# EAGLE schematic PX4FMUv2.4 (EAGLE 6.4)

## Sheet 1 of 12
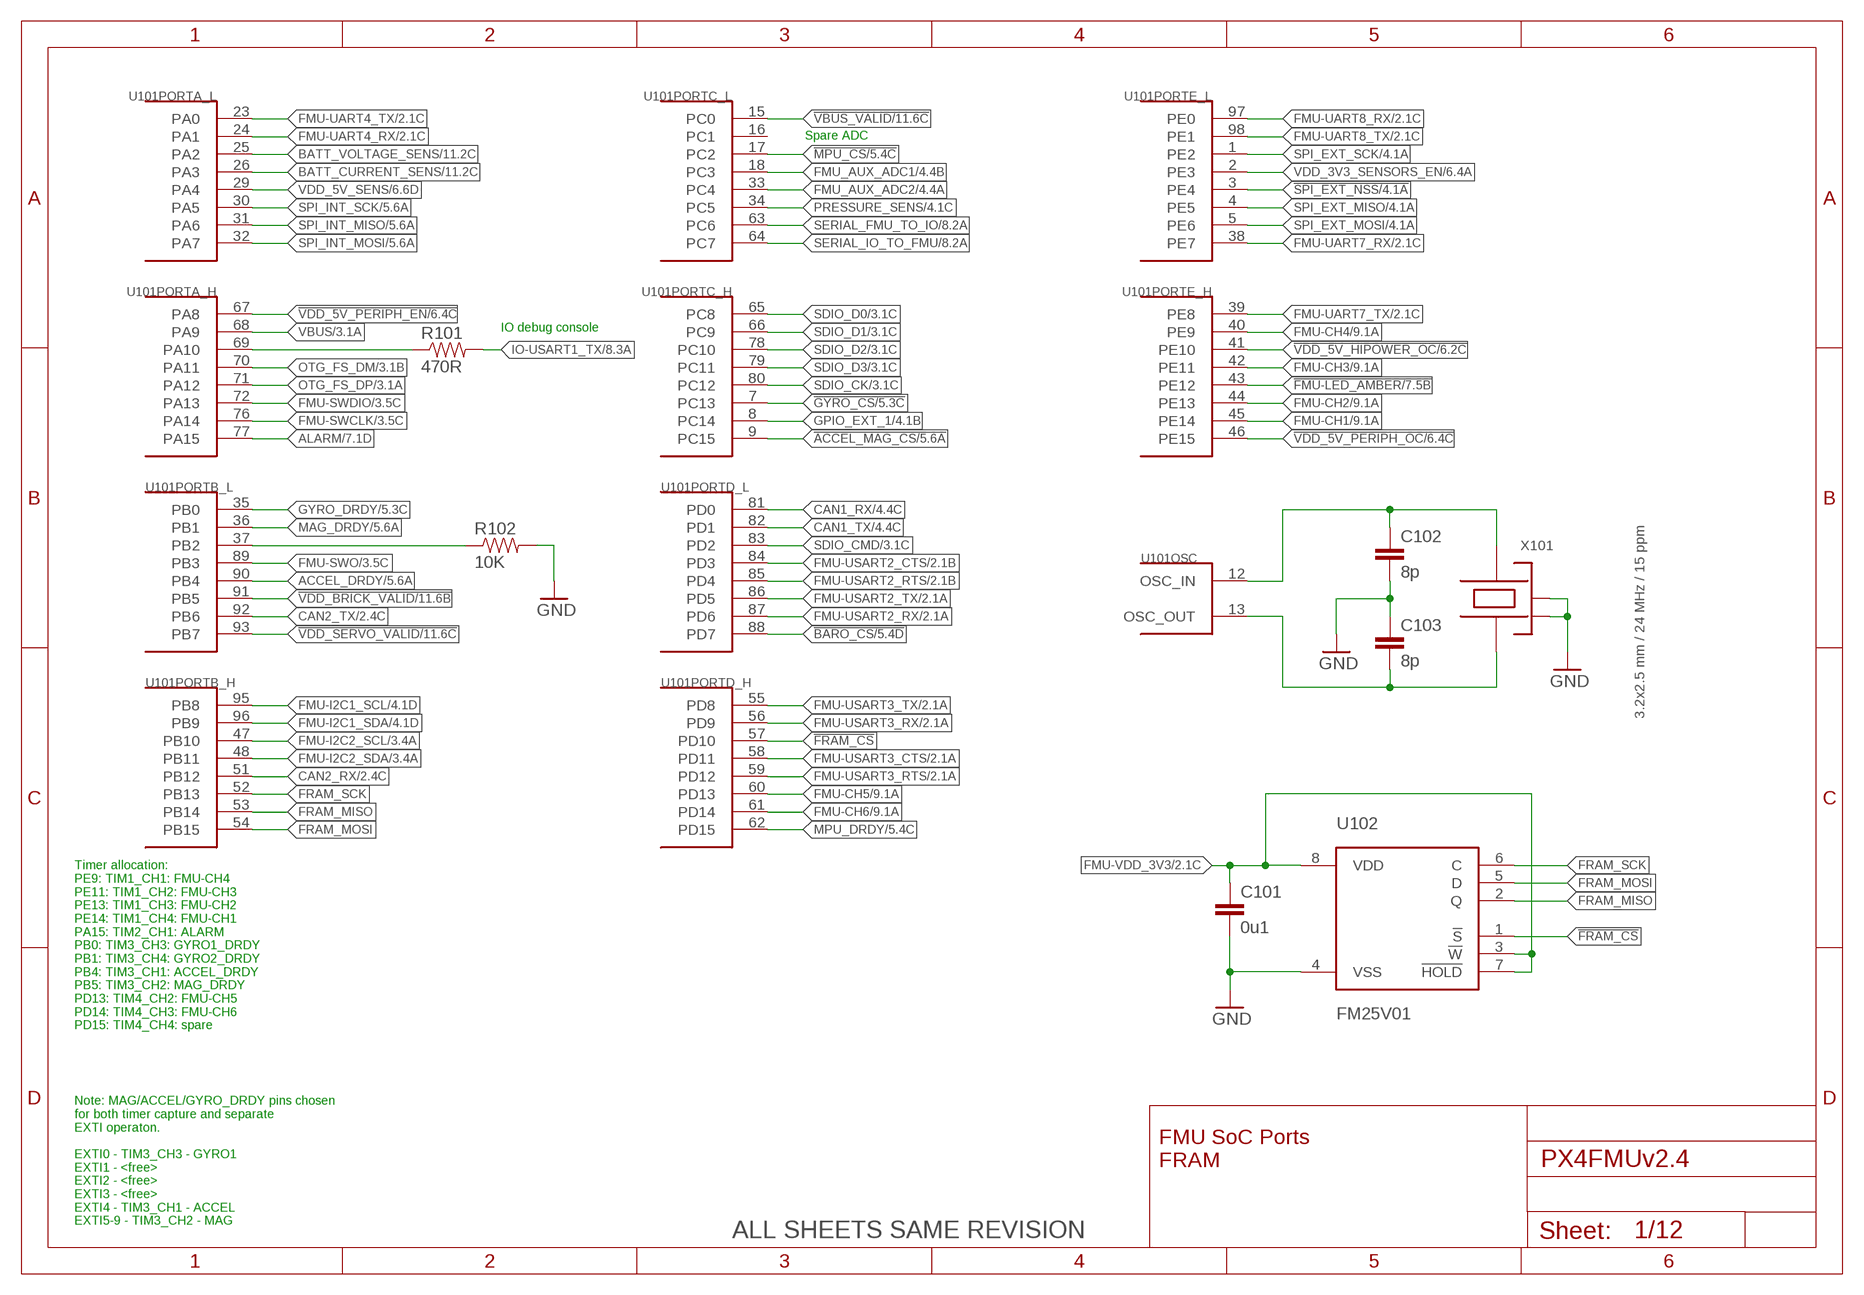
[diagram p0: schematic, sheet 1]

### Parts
C101  0u1  CAP0402  [0402-CAP]
C102  8p  CAP0402  [0402-CAP]
C103  8p  CAP0402  [0402-CAP]
R101  470R  RESISTOR0402-RES  [0402-RES]
R102  10K  RESISTOR0402-RES  [0402-RES]
U101  STM32F4X7VX  [TQFP100]
U102  FM25V01  [SO08]
X101  3.2x2.5 mm / 24 MHz / 15 ppm  OSCILLATOR-3.2X2.5  [OSCILLATOR-3.2X2.5]

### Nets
!ACCEL_MAG_CS: U101.9(PORTC_H:PC15) ; also sheet 5
!BARO_CS: U101.88(PORTD_L:PD7) ; also sheet 5
!FMU-LED_AMBER: U101.43(PORTE_H:PE12) ; also sheet 7
!FRAM_CS: U101.57(PORTD_H:PD10) U102.1(!S)
!GYRO_CS: U101.7(PORTC_H:PC13) ; also sheet 5
!MPU_CS: U101.17(PORTC_L:PC2) ; also sheet 5
!SPI_EXT_NSS: U101.3(PORTE_L:PE4) ; also sheet 4
!VBUS_VALID: U101.15(PORTC_L:PC0) ; also sheet 11,12
!VDD_5V_HIPOWER_OC: U101.41(PORTE_H:PE10) ; also sheet 6
!VDD_5V_PERIPH_EN: U101.67(PORTA_H:PA8) ; also sheet 6
!VDD_5V_PERIPH_OC: U101.46(PORTE_H:PE15) ; also sheet 6
!VDD_BRICK_VALID: U101.91(PORTB_L:PB5) ; also sheet 11,12
!VDD_SERVO_VALID: U101.93(PORTB_L:PB7) ; also sheet 11,12
ACCEL_DRDY: U101.90(PORTB_L:PB4) ; also sheet 5
ALARM: U101.77(PORTA_H:PA15) ; also sheet 7
BATT_CURRENT_SENS: U101.26(PORTA_L:PA3) ; also sheet 11
BATT_VOLTAGE_SENS: U101.25(PORTA_L:PA2) ; also sheet 11
CAN1_RX: U101.81(PORTD_L:PD0) ; also sheet 4
CAN1_TX: U101.82(PORTD_L:PD1) ; also sheet 4
CAN2_RX: U101.51(PORTB_H:PB12) ; also sheet 2
CAN2_TX: U101.92(PORTB_L:PB6) ; also sheet 2
FMU-CH1: U101.45(PORTE_H:PE14) ; also sheet 9
FMU-CH2: U101.44(PORTE_H:PE13) ; also sheet 9
FMU-CH3: U101.42(PORTE_H:PE11) ; also sheet 9
FMU-CH4: U101.40(PORTE_H:PE9) ; also sheet 9
FMU-CH5: U101.60(PORTD_H:PD13) ; also sheet 9
FMU-CH6: U101.61(PORTD_H:PD14) ; also sheet 9
FMU-I2C1_SCL: U101.95(PORTB_H:PB8) ; also sheet 4
FMU-I2C1_SDA: U101.96(PORTB_H:PB9) ; also sheet 4
FMU-I2C2_SCL: U101.47(PORTB_H:PB10) ; also sheet 3,7
FMU-I2C2_SDA: U101.48(PORTB_H:PB11) ; also sheet 3,7
FMU-SWCLK: U101.76(PORTA_H:PA14) ; also sheet 3
FMU-SWDIO: U101.72(PORTA_H:PA13) ; also sheet 3
FMU-SWO: U101.89(PORTB_L:PB3) ; also sheet 3
FMU-UART4_RX: U101.24(PORTA_L:PA1) ; also sheet 2
FMU-UART4_TX: U101.23(PORTA_L:PA0) ; also sheet 2
FMU-UART7_RX: U101.38(PORTE_L:PE7) ; also sheet 2
FMU-UART7_TX: U101.39(PORTE_H:PE8) ; also sheet 2
FMU-UART8_RX: U101.97(PORTE_L:PE0) ; also sheet 2
FMU-UART8_TX: U101.98(PORTE_L:PE1) ; also sheet 2
FMU-USART2_CTS: U101.84(PORTD_L:PD3) ; also sheet 2
FMU-USART2_RTS: U101.85(PORTD_L:PD4) ; also sheet 2
FMU-USART2_RX: U101.87(PORTD_L:PD6) ; also sheet 2
FMU-USART2_TX: U101.86(PORTD_L:PD5) ; also sheet 2
FMU-USART3_CTS: U101.58(PORTD_H:PD11) ; also sheet 2
FMU-USART3_RTS: U101.59(PORTD_H:PD12) ; also sheet 2
FMU-USART3_RX: U101.56(PORTD_H:PD9) ; also sheet 2
FMU-USART3_TX: U101.55(PORTD_H:PD8) ; also sheet 2
FMU-VDD_3V3 [power]: C101.P$1 U102.3(!W) U102.7(!HOLD) U102.8(VDD) ; also sheet 2,3,4,6,7,9,12
FMU_AUX_ADC1: U101.18(PORTC_L:PC3) ; also sheet 4
FMU_AUX_ADC2: U101.33(PORTC_L:PC4) ; also sheet 4
FRAM_MISO: U101.53(PORTB_H:PB14) U102.2(Q)
FRAM_MOSI: U101.54(PORTB_H:PB15) U102.5(D)
FRAM_SCK: U101.52(PORTB_H:PB13) U102.6(C)
GND [power]: C101.P$2 C102.P$2 C103.P$1 R102.P$2 U102.4(VSS) X101.2(NC_2) X101.4(NC_4) ; also sheet 2,3,4,5,6,7,8,9,10,11,12
GPIO_EXT_1: U101.8(PORTC_H:PC14) ; also sheet 4
GYRO_DRDY: U101.35(PORTB_L:PB0) ; also sheet 5
IO-USART1_TX: R101.P$2 ; also sheet 8
MAG_DRDY: U101.36(PORTB_L:PB1) ; also sheet 5
MPU_DRDY [power]: U101.62(PORTD_H:PD15) ; also sheet 5
N$1: C103.P$2 U101.13(OSC:OSC_OUT) X101.1
N$2: C102.P$1 U101.12(OSC:OSC_IN) X101.3
N$23: R101.P$1 U101.69(PORTA_H:PA10)
OTG_FS_DM: U101.70(PORTA_H:PA11) ; also sheet 3
OTG_FS_DP: U101.71(PORTA_H:PA12) ; also sheet 3
PB2-BOOT1: R102.P$1 U101.37(PORTB_L:PB2)
PRESSURE_SENS: U101.34(PORTC_L:PC5) ; also sheet 4
SDIO_CK: U101.80(PORTC_H:PC12) ; also sheet 3
SDIO_CMD: U101.83(PORTD_L:PD2) ; also sheet 3
SDIO_D0: U101.65(PORTC_H:PC8) ; also sheet 3
SDIO_D1: U101.66(PORTC_H:PC9) ; also sheet 3
SDIO_D2: U101.78(PORTC_H:PC10) ; also sheet 3
SDIO_D3: U101.79(PORTC_H:PC11) ; also sheet 3
SERIAL_FMU_TO_IO: U101.63(PORTC_L:PC6) ; also sheet 8
SERIAL_IO_TO_FMU: U101.64(PORTC_L:PC7) ; also sheet 8
SPI_EXT_MISO: U101.4(PORTE_L:PE5) ; also sheet 4
SPI_EXT_MOSI: U101.5(PORTE_L:PE6) ; also sheet 4
SPI_EXT_SCK: U101.1(PORTE_L:PE2) ; also sheet 4
SPI_INT_MISO: U101.31(PORTA_L:PA6) ; also sheet 5
SPI_INT_MOSI: U101.32(PORTA_L:PA7) ; also sheet 5
SPI_INT_SCK: U101.30(PORTA_L:PA5) ; also sheet 5
VBUS [power]: U101.68(PORTA_H:PA9) ; also sheet 3,11,12
VDD_3V3_SENSORS_EN: U101.2(PORTE_L:PE3) ; also sheet 6
VDD_5V_SENS: U101.29(PORTA_L:PA4) ; also sheet 6
Unconnected: U101.16(PORTC_L:PC1)

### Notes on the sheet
- Spare ADC
- IO debug console
- Timer allocation:
  PE9: TIM1_CH1: FMU-CH4
  PE11: TIM1_CH2: FMU-CH3
  PE13: TIM1_CH3: FMU-CH2
  PE14: TIM1_CH4: FMU-CH1
  PA15: TIM2_CH1: ALARM
  PB0: TIM3_CH3: GYRO1_DRDY
  PB1: TIM3_CH4: GYRO2_DRDY
  PB4: TIM3_CH1: ACCEL_DRDY
  PB5: TIM3_CH2: MAG_DRDY
  PD13: TIM4_CH2: FMU-CH5
  PD14: TIM4_CH3: FMU-CH6
  PD15: TIM4_CH4: spare
- FMU SoC Ports
  FRAM
- Note: MAG/ACCEL/GYRO_DRDY pins chosen
  for both timer capture and separate
  EXTI operaton.
  
  EXTI0 - TIM3_CH3 - GYRO1
  EXTI1 - <free>
  EXTI2 - <free>
  EXTI3 - <free>
  EXTI4 - TIM3_CH1 - ACCEL
  EXTI5-9 - TIM3_CH2 - MAG
- ALL SHEETS SAME REVISION

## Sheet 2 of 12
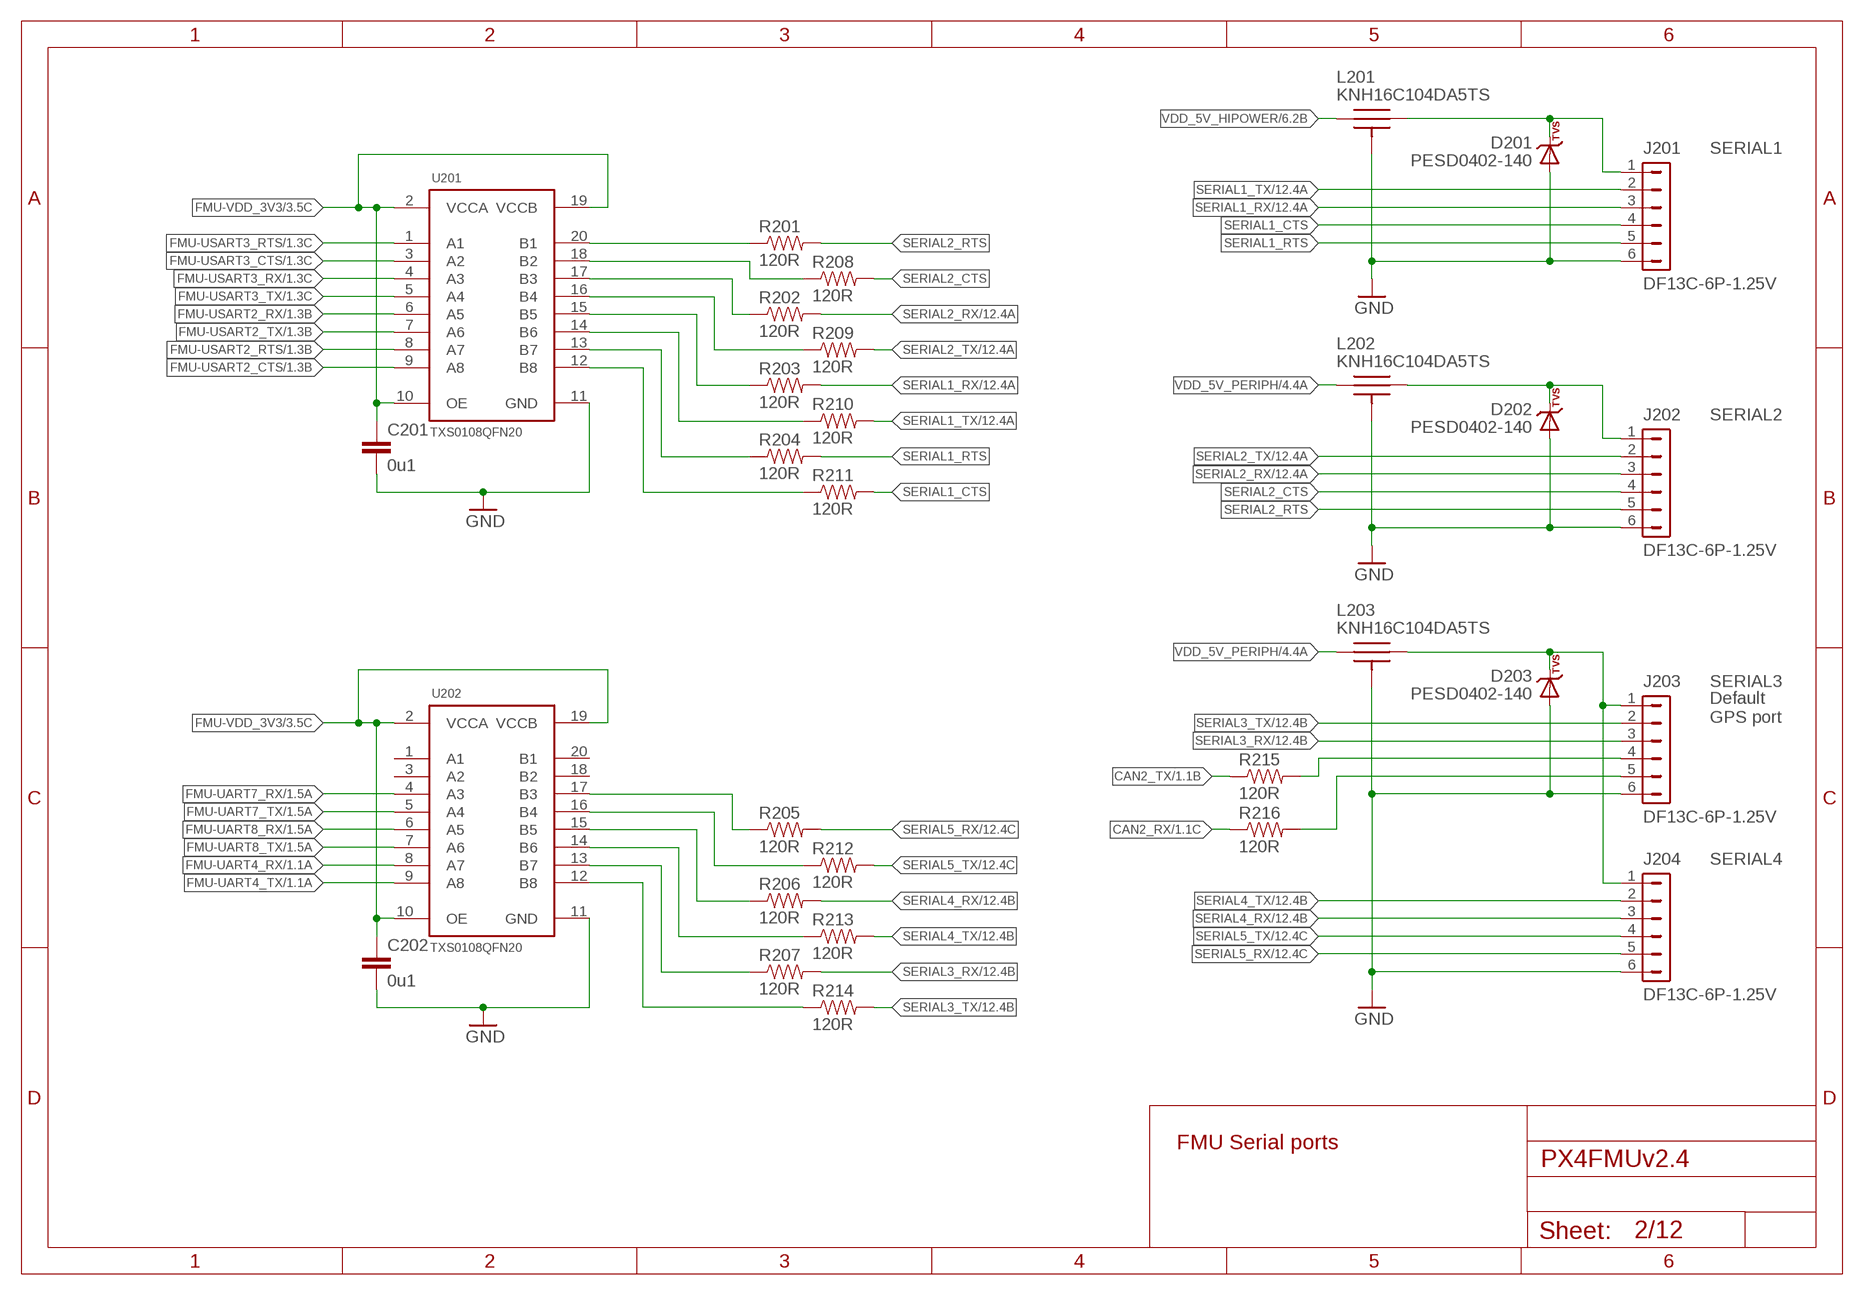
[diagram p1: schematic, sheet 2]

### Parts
C201  0u1  CAP0402  [0402-CAP]
C202  0u1  CAP0402  [0402-CAP]
D201  PESD0402-140  DIODE-TVS  [0402-TVS]
D202  PESD0402-140  DIODE-TVS  [0402-TVS]
D203  PESD0402-140  DIODE-TVS  [0402-TVS]
J201  DF13C-6P-1.25V  DF13-6P-1.25V  [DF13C-6P-1.25V]
J202  DF13C-6P-1.25V  DF13-6P-1.25V  [DF13C-6P-1.25V]
J203  DF13C-6P-1.25V  DF13-6P-1.25V  [DF13C-6P-1.25V]
J204  DF13C-6P-1.25V  DF13-6P-1.25V  [DF13C-6P-1.25V]
L201  KNH16C104DA5TS  [KYOCERA-KNH16-DA]
L202  KNH16C104DA5TS  [KYOCERA-KNH16-DA]
L203  KNH16C104DA5TS  [KYOCERA-KNH16-DA]
R201  120R  RESISTOR0402-RES  [0402-RES]
R202  120R  RESISTOR0402-RES  [0402-RES]
R203  120R  RESISTOR0402-RES  [0402-RES]
R204  120R  RESISTOR0402-RES  [0402-RES]
R205  120R  RESISTOR0402-RES  [0402-RES]
R206  120R  RESISTOR0402-RES  [0402-RES]
R207  120R  RESISTOR0402-RES  [0402-RES]
R208  120R  RESISTOR0402-RES  [0402-RES]
R209  120R  RESISTOR0402-RES  [0402-RES]
R210  120R  RESISTOR0402-RES  [0402-RES]
R211  120R  RESISTOR0402-RES  [0402-RES]
R212  120R  RESISTOR0402-RES  [0402-RES]
R213  120R  RESISTOR0402-RES  [0402-RES]
R214  120R  RESISTOR0402-RES  [0402-RES]
R215  120R  RESISTOR0402-RES  [0402-RES]
R216  120R  RESISTOR0402-RES  [0402-RES]
U201  TXS0108QFN20  [QFN20-RGY]
U202  TXS0108QFN20  [QFN20-RGY]

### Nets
CAN2_RX: R216.P$1 ; also sheet 1
CAN2_TX: R215.P$1 ; also sheet 1
FMU-UART4_RX: U202.8(A7) ; also sheet 1
FMU-UART4_TX: U202.9(A8) ; also sheet 1
FMU-UART7_RX: U202.4(A3) ; also sheet 1
FMU-UART7_TX: U202.5(A4) ; also sheet 1
FMU-UART8_RX: U202.6(A5) ; also sheet 1
FMU-UART8_TX: U202.7(A6) ; also sheet 1
FMU-USART2_CTS: U201.9(A8) ; also sheet 1
FMU-USART2_RTS: U201.8(A7) ; also sheet 1
FMU-USART2_RX: U201.6(A5) ; also sheet 1
FMU-USART2_TX: U201.7(A6) ; also sheet 1
FMU-USART3_CTS: U201.3(A2) ; also sheet 1
FMU-USART3_RTS: U201.1(A1) ; also sheet 1
FMU-USART3_RX: U201.4(A3) ; also sheet 1
FMU-USART3_TX: U201.5(A4) ; also sheet 1
FMU-VDD_3V3 [power]: C201.P$1 C202.P$1 U201.2(VCCA) U201.10(OE) U201.19(VCCB) U202.2(VCCA) U202.10(OE) U202.19(VCCB) ; also sheet 1,3,4,6,7,9,12
GND [power]: C201.P$2 C202.P$2 D201.A D202.A D203.A J201.6 J202.6 J203.6 J204.6 L201.P$3 L201.P$4 L201.P$5 L202.P$3 L202.P$4 L202.P$5 L203.P$3 L203.P$4 L203.P$5 U201.11(GND) U202.11(GND) ; also sheet 1,3,4,5,6,7,8,9,10,11,12
N$5 [power]: D201.C J201.1 L201.P$2
N$14: J203.4 R215.P$2
N$19: J203.5 R216.P$2
N$70: R201.P$1 U201.20(B1)
N$82: R208.P$1 U201.18(B2)
N$83: R202.P$1 U201.17(B3)
N$84: R209.P$1 U201.16(B4)
N$85: R203.P$1 U201.15(B5)
N$86: R210.P$1 U201.14(B6)
N$87: R204.P$1 U201.13(B7)
N$88: R211.P$1 U201.12(B8)
N$89: R207.P$1 U202.13(B7)
N$90: R214.P$1 U202.12(B8)
N$91: R205.P$1 U202.17(B3)
N$92: R212.P$1 U202.16(B4)
N$93: R206.P$1 U202.15(B5)
N$94: R213.P$1 U202.14(B6)
N$100 [power]: D203.C J203.1 J204.1 L203.P$2
N$101 [power]: D202.C J202.1 L202.P$2
SERIAL1_CTS: J201.4 R211.P$2
SERIAL1_RTS: J201.5 R204.P$2
SERIAL1_RX: J201.3 R203.P$2 ; also sheet 12
SERIAL1_TX: J201.2 R210.P$2 ; also sheet 12
SERIAL2_CTS: J202.4 R208.P$2
SERIAL2_RTS: J202.5 R201.P$2
SERIAL2_RX: J202.3 R202.P$2 ; also sheet 12
SERIAL2_TX: J202.2 R209.P$2 ; also sheet 12
SERIAL3_RX: J203.3 R207.P$2 ; also sheet 12
SERIAL3_TX: J203.2 R214.P$2 ; also sheet 12
SERIAL4_RX: J204.3 R206.P$2 ; also sheet 12
SERIAL4_TX: J204.2 R213.P$2 ; also sheet 12
SERIAL5_RX: J204.5 R205.P$2 ; also sheet 12
SERIAL5_TX: J204.4 R212.P$2 ; also sheet 12
VDD_5V_HIPOWER [power]: L201.P$1 ; also sheet 6
VDD_5V_PERIPH [power]: L202.P$1 L203.P$1 ; also sheet 4,6
Unconnected: U202.1(A1) U202.3(A2) U202.18(B2) U202.20(B1)

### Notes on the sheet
- SERIAL1
- SERIAL2
- SERIAL3
- Default 
  GPS port
- SERIAL4
- FMU Serial ports

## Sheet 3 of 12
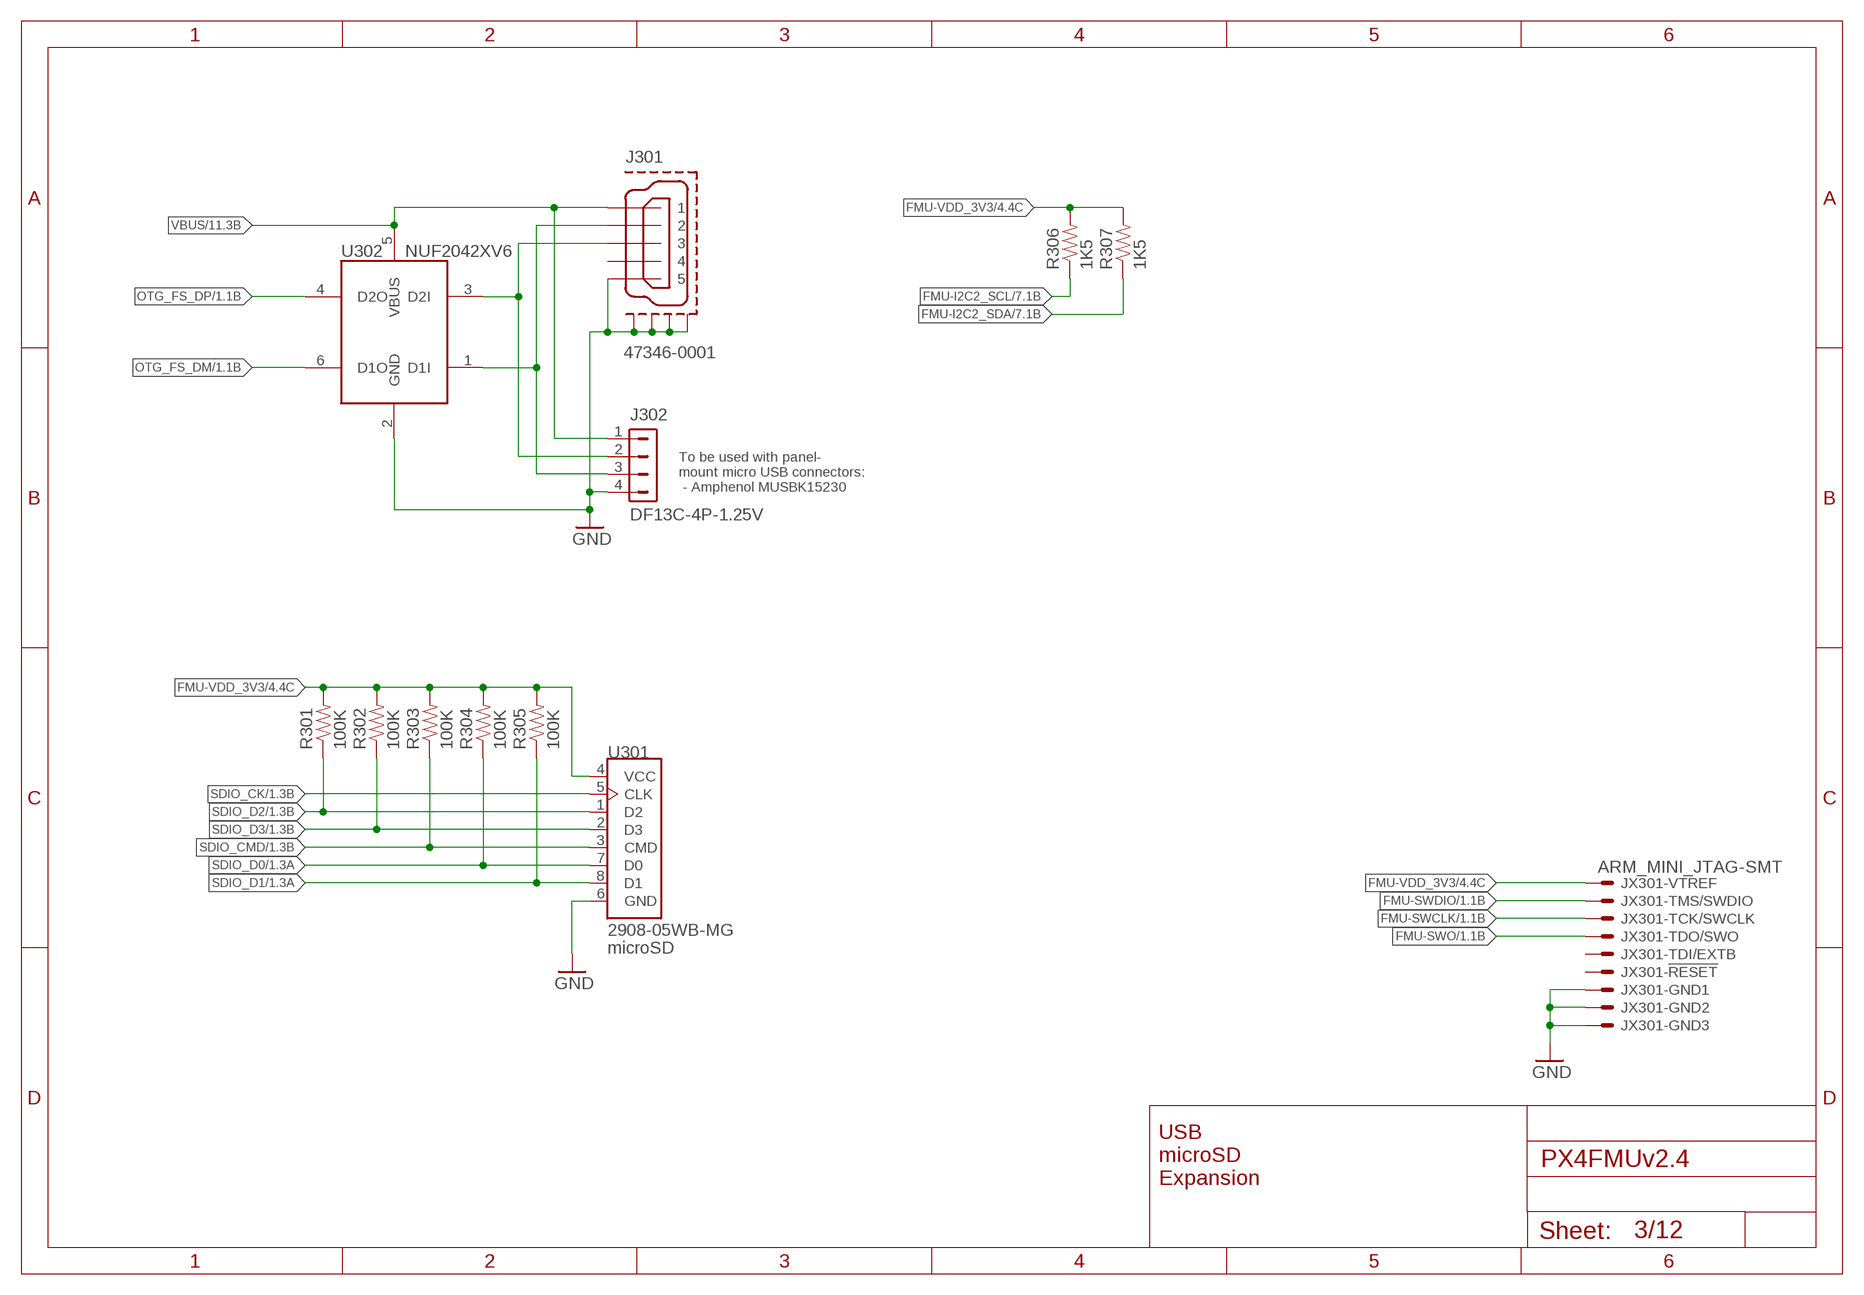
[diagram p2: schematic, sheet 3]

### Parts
J301  47346-0001  MOLEX-47346-0001  [MOLEX-47346-0001]
J302  DF13C-4P-1.25V  DF13-4P-1.25V  [DF13C-4P-1.25V]
JX301  ARM_MINI_JTAG-SMT  [FTSH-105-01-XXX-DV-K]
R301  100K  RESISTOR0402-RES  [0402-RES]
R302  100K  RESISTOR0402-RES  [0402-RES]
R303  100K  RESISTOR0402-RES  [0402-RES]
R304  100K  RESISTOR0402-RES  [0402-RES]
R305  100K  RESISTOR0402-RES  [0402-RES]
R306  1K5  RESISTOR0402-RES  [0402-RES]
R307  1K5  RESISTOR0402-RES  [0402-RES]
U301  2908-05WB-MG  MICROSDSDI  [MICROSD]
U302  NUF2042XV6  [SOT563-6]

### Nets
FMU-I2C2_SCL: R306.P$1 ; also sheet 1,7
FMU-I2C2_SDA: R307.P$1 ; also sheet 1,7
FMU-SWCLK: JX301.4 ; also sheet 1
FMU-SWDIO: JX301.2 ; also sheet 1
FMU-SWO: JX301.6 ; also sheet 1
FMU-VDD_3V3 [power]: JX301.1 R301.P$2 R302.P$2 R303.P$2 R304.P$2 R305.P$2 R306.P$2 R307.P$2 U301.4(VCC) ; also sheet 1,2,4,6,7,9,12
GND [power]: J301.GND J301.GND1 J301.GND2 J301.GND3 J301.GND4 J302.4 JX301.3 JX301.5 JX301.9 U301.6(GND) U302.2(GND) ; also sheet 1,2,4,5,6,7,8,9,10,11,12
OTG_DM1: J301.D- J302.3 U302.1(D1I)
OTG_DP1: J301.D+ J302.2 U302.3(D2I)
OTG_FS_DM: U302.6(D1O) ; also sheet 1
OTG_FS_DP: U302.4(D2O) ; also sheet 1
SDIO_CK: U301.5(CLK) ; also sheet 1
SDIO_CMD: R303.P$1 U301.3(CMD) ; also sheet 1
SDIO_D0: R304.P$1 U301.7(D0) ; also sheet 1
SDIO_D1: R305.P$1 U301.8(D1) ; also sheet 1
SDIO_D2: R301.P$1 U301.1(D2) ; also sheet 1
SDIO_D3: R302.P$1 U301.2(D3) ; also sheet 1
VBUS [power]: J301.VBUS J302.1 U302.5(VBUS) ; also sheet 1,11,12
Unconnected: J301.ID JX301.8 JX301.10

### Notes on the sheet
- To be used with panel-
  mount micro USB connectors:
   - Amphenol MUSBK15230
- microSD
- USB
  microSD
  Expansion

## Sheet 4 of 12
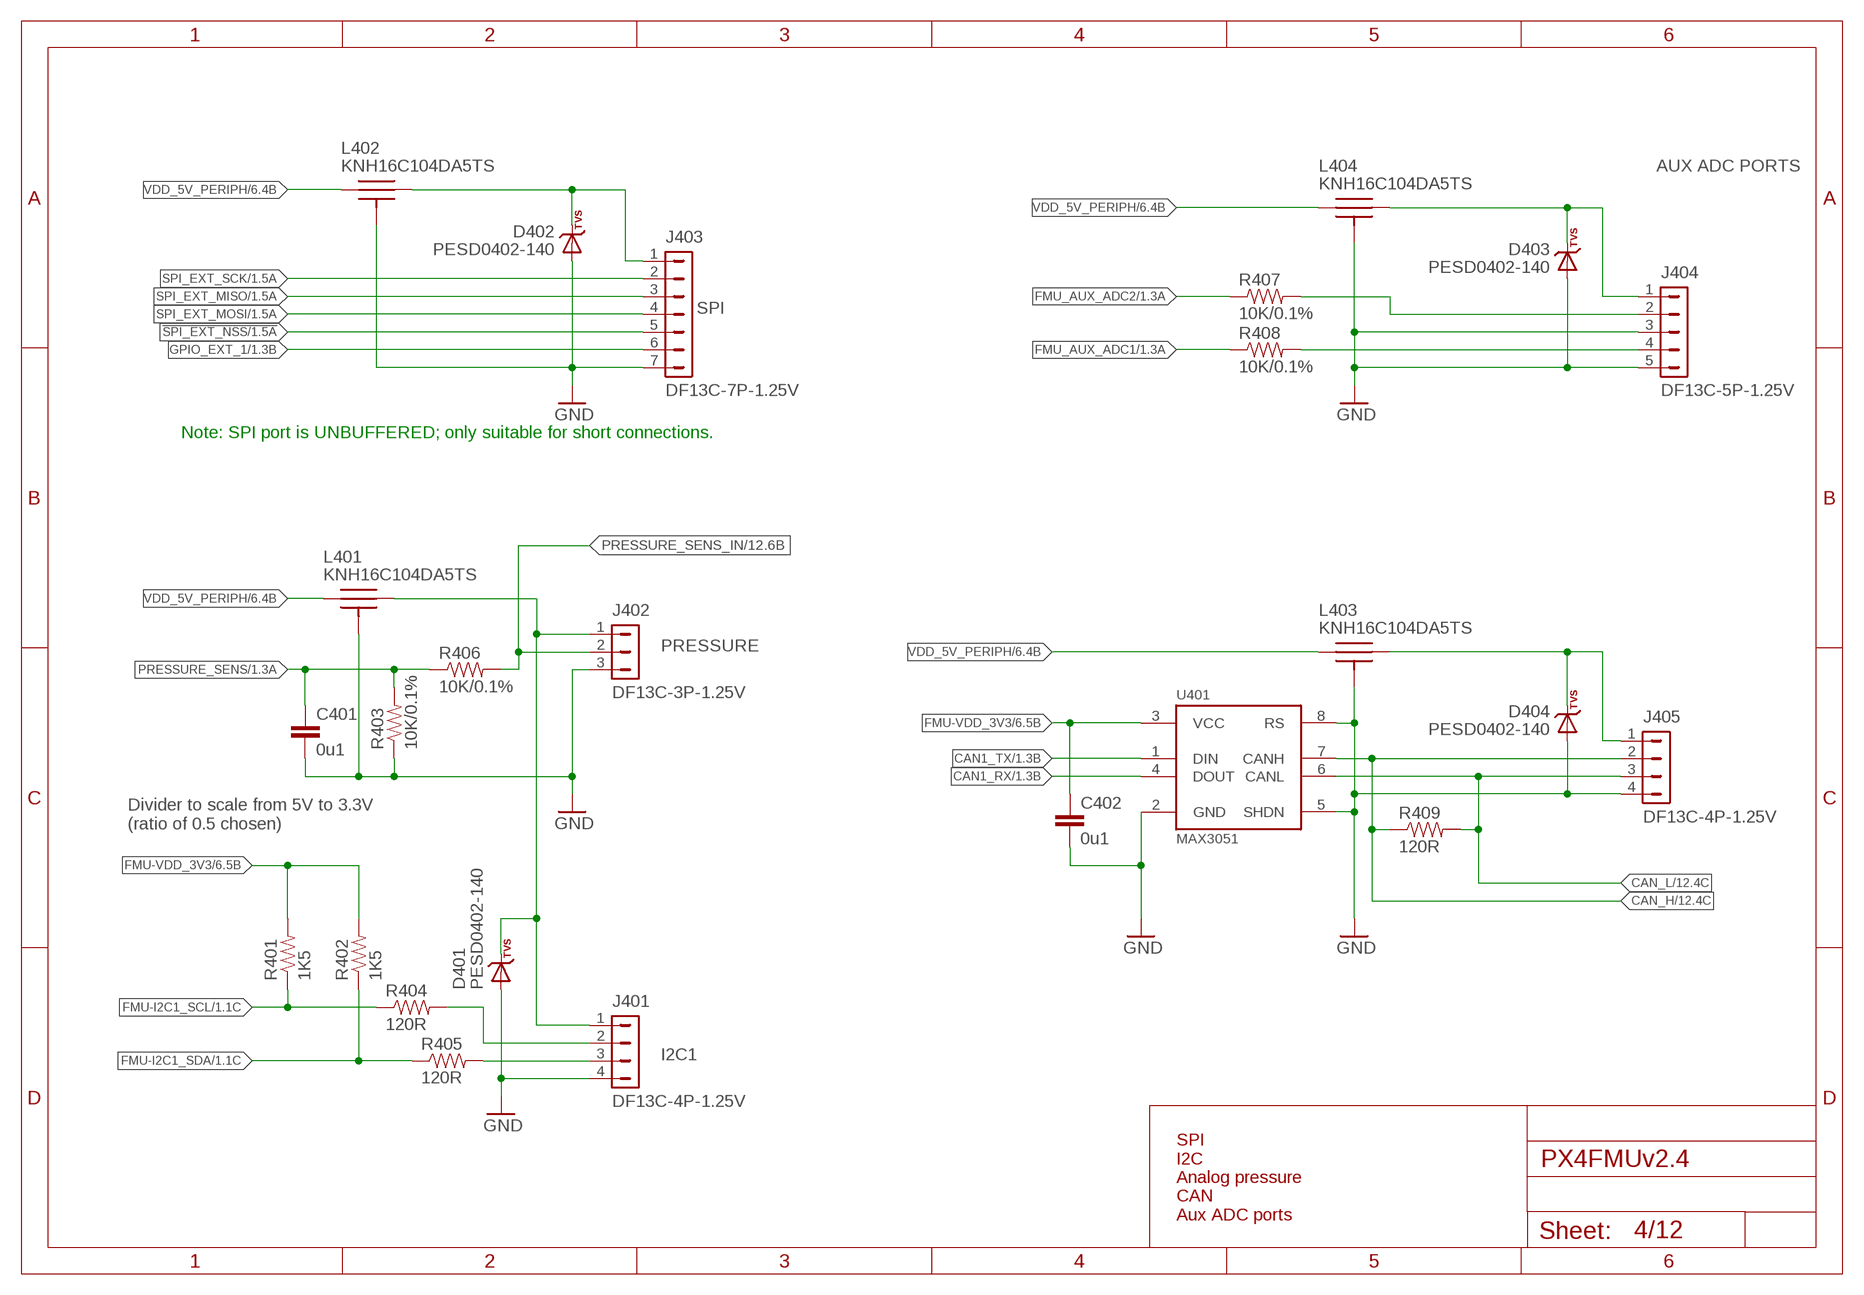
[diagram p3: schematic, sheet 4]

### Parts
C401  0u1  CAP0402  [0402-CAP]
C402  0u1  CAP0402  [0402-CAP]
D401  PESD0402-140  DIODE-TVS  [0402-TVS]
D402  PESD0402-140  DIODE-TVS  [0402-TVS]
D403  PESD0402-140  DIODE-TVS  [0402-TVS]
D404  PESD0402-140  DIODE-TVS  [0402-TVS]
J401  DF13C-4P-1.25V  DF13-4P-1.25V  [DF13C-4P-1.25V]
J402  DF13C-3P-1.25V  DF13-3P-1.25V  [DF13C-3P-1.25V]
J403  DF13C-7P-1.25V  DF13-7P-1.25V  [DF13C-7P-1.25V]
J404  DF13C-5P-1.25V  DF13-5P-1.25V  [DF13C-5P-1.25V]
J405  DF13C-4P-1.25V  DF13-4P-1.25V  [DF13C-4P-1.25V]
L401  KNH16C104DA5TS  [KYOCERA-KNH16-DA]
L402  KNH16C104DA5TS  [KYOCERA-KNH16-DA]
L403  KNH16C104DA5TS  [KYOCERA-KNH16-DA]
L404  KNH16C104DA5TS  [KYOCERA-KNH16-DA]
R401  1K5  RESISTOR0402-RES  [0402-RES]
R402  1K5  RESISTOR0402-RES  [0402-RES]
R403  10K/0.1%  RESISTOR0402-RES  [0402-RES]
R404  120R  RESISTOR0402-RES  [0402-RES]
R405  120R  RESISTOR0402-RES  [0402-RES]
R406  10K/0.1%  RESISTOR0402-RES  [0402-RES]
R407  10K/0.1%  RESISTOR0402-RES  [0402-RES]
R408  10K/0.1%  RESISTOR0402-RES  [0402-RES]
R409  120R  RESISTOR0402-RES  [0402-RES]
U401  MAX3051  MAX3051MAX3051EKA  [SOT23-8]

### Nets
!SPI_EXT_NSS: J403.5 ; also sheet 1
CAN1_RX: U401.4(DOUT) ; also sheet 1
CAN1_TX: U401.1(DIN) ; also sheet 1
CAN_H: J405.2 R409.P$1 U401.7(CANH) ; also sheet 12
CAN_L: J405.3 R409.P$2 U401.6(CANL) ; also sheet 12
FMU-I2C1_SCL: R401.P$1 R404.P$1 ; also sheet 1
FMU-I2C1_SDA: R402.P$1 R405.P$1 ; also sheet 1
FMU-VDD_3V3 [power]: C402.P$1 R401.P$2 R402.P$2 U401.3(VCC) ; also sheet 1,2,3,6,7,9,12
FMU_AUX_ADC1: R408.P$1 ; also sheet 1
FMU_AUX_ADC1_PROT: J404.4 R408.P$2
FMU_AUX_ADC2: R407.P$1 ; also sheet 1
FMU_AUX_ADC2_PROT: J404.2 R407.P$2
GND [power]: C401.P$2 C402.P$2 D401.A D402.A D403.A D404.A J401.4 J402.3 J403.7 J404.3 J404.5 J405.4 L401.P$3 L401.P$4 L401.P$5 L402.P$3 L402.P$4 L402.P$5 L403.P$3 L403.P$4 L403.P$5 L404.P$3 L404.P$4 L404.P$5 R403.P$1 U401.2(GND) U401.5(SHDN) U401.8(RS) ; also sheet 1,2,3,5,6,7,8,9,10,11,12
GPIO_EXT_1: J403.6 ; also sheet 1
N$33: J401.2 R404.P$2
N$37: J401.3 R405.P$2
N$41 [power]: D402.C J403.1 L402.P$2
N$42 [power]: D401.C J401.1 J402.1 L401.P$2
N$48 [power]: D404.C J405.1 L403.P$2
N$98 [power]: D403.C J404.1 L404.P$2
PRESSURE_SENS: C401.P$1 R403.P$2 R406.P$1 ; also sheet 1
PRESSURE_SENS_IN: J402.2 R406.P$2 ; also sheet 12
SPI_EXT_MISO: J403.3 ; also sheet 1
SPI_EXT_MOSI: J403.4 ; also sheet 1
SPI_EXT_SCK: J403.2 ; also sheet 1
VDD_5V_PERIPH [power]: L401.P$1 L402.P$1 L403.P$1 L404.P$1 ; also sheet 2,6

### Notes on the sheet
- AUX ADC PORTS
- SPI
- Note: SPI port is UNBUFFERED; only suitable for short connections.
- PRESSURE
- Divider to scale from 5V to 3.3V
  (ratio of 0.5 chosen)
- I2C1
- SPI
  I2C
  Analog pressure
  CAN
  Aux ADC ports

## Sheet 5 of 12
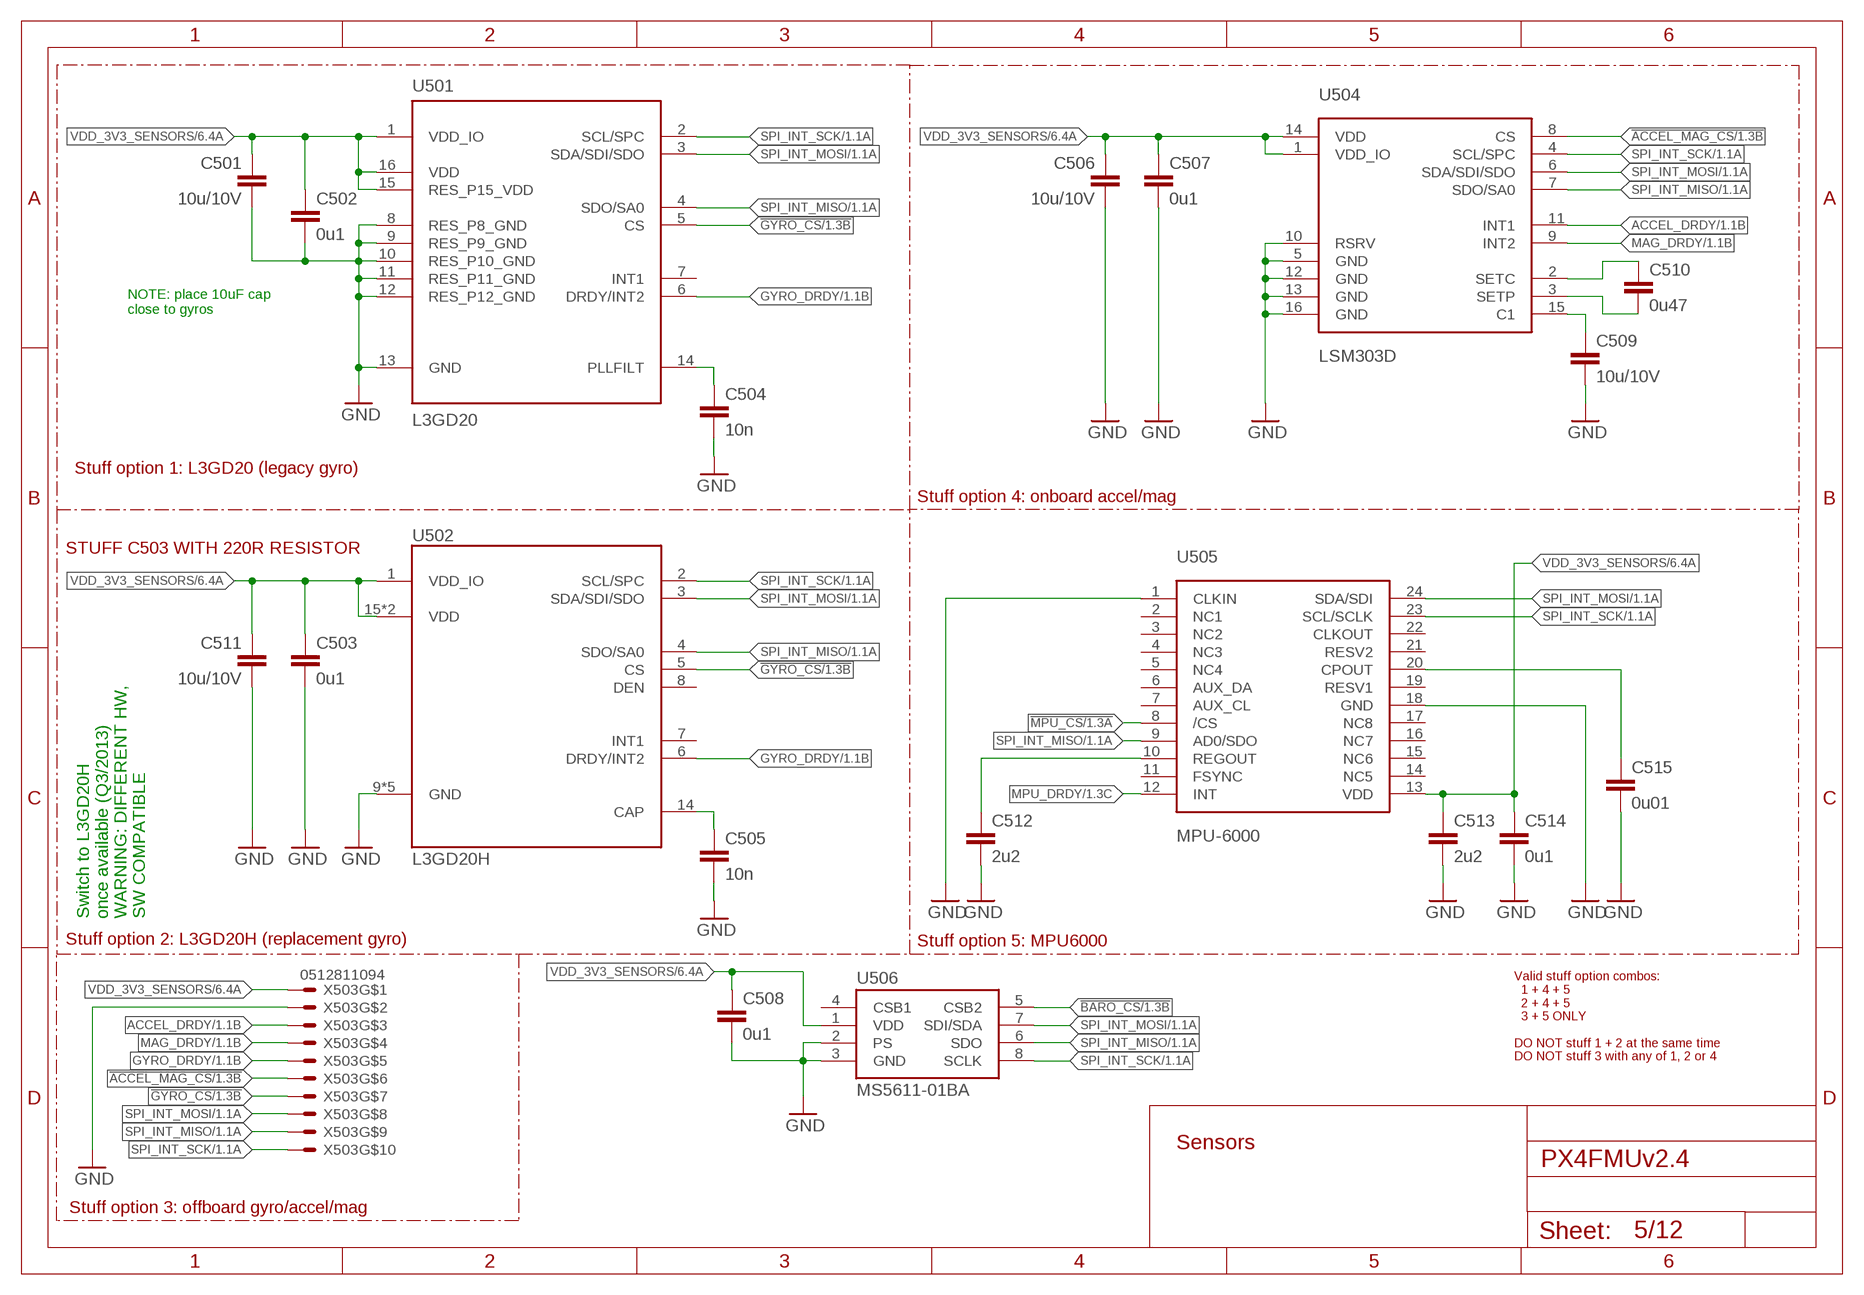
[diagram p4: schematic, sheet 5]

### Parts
C501  10u/10V  CAP0805  [0805-CAP]
C502  0u1  CAP0402  [0402-CAP]
C503  0u1  CAP0402  [0402-CAP]
C504  10n  CAP0402  [0402-CAP]
C505  10n  CAP0402  [0402-CAP]
C506  10u/10V  CAP0805  [0805-CAP]
C507  0u1  CAP0402  [0402-CAP]
C508  0u1  CAP0402  [0402-CAP]
C509  10u/10V  CAP0805  [0805-CAP]
C510  0u47  CAP0402  [0402-CAP]
C511  10u/10V  CAP0805  [0805-CAP]
C512  2u2  CAP0603  [0603-CAP]
C513  2u2  CAP0603  [0603-CAP]
C514  0u1  CAP0402  [0402-CAP]
C515  0u01  CAP0603  [0603-CAP]
U501  L3GD20  L3G4200DH-LL  [L3G4200DH-MAN]
U502  L3GD20H  [LGA-16L]
U504  LSM303D  [LGA-16L]
U505  MPU-6000  [QFN-24]
U506  MS5611-01BA  [MS5611-01BA]
X503  0512811094  CONN_FPC_10RA  [51281-1094]

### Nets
!ACCEL_MAG_CS: U504.8(CS) X503.6 ; also sheet 1
!BARO_CS: U506.5(CSB2) ; also sheet 1
!GYRO_CS: U501.5(CS) U502.5(CS) X503.7 ; also sheet 1
!MPU_CS: U505.8(/CS) ; also sheet 1
ACCEL_DRDY: U504.11(INT1) X503.3 ; also sheet 1
GND [power]: C501.P$2 C502.P$2 C503.P$2 C504.P$2 C505.P$2 C506.P$2 C507.P$2 C508.P$2 C509.P$2 C511.P$2 C512.P$2 C513.P$2 C514.P$2 C515.P$2 U501.8(RES_P8_GND) U501.9(RES_P9_GND) U501.10(RES_P10_GND) U501.11(RES_P11_GND) U501.12(RES_P12_GND) U501.13(GND) U502.9(GND) U502.10(GND) U502.11(GND) U502.12(GND) U502.13(GND) U504.5(GND) U504.10(RSRV) U504.12(GND) U504.13(GND) U504.16(GND) U505.1(CLKIN) U505.18(GND) U506.2(PS) U506.3(GND) X503.2 ; also sheet 1,2,3,4,6,7,8,9,10,11,12
GYRO_DRDY: U501.6(DRDY/INT2) U502.6(DRDY/INT2) X503.5 ; also sheet 1
MAG_DRDY: U504.9(INT2) X503.4 ; also sheet 1
MPU_DRDY [power]: U505.12(INT) ; also sheet 1
N$6: C509.P$1 U504.15(C1)
N$10: C510.P$1 U504.2(SETC)
N$17: C510.P$2 U504.3(SETP)
N$30: C505.P$1 U502.14(CAP)
N$35: C504.P$1 U501.14(PLLFILT)
N$50: C512.P$1 U505.10(REGOUT)
N$51: C515.P$1 U505.20(CPOUT)
SPI_INT_MISO: U501.4(SDO/SA0) U502.4(SDO/SA0) U504.7(SDO/SA0) U505.9(AD0/SDO) U506.6(SDO) X503.9 ; also sheet 1
SPI_INT_MOSI: U501.3(SDA/SDI/SDO) U502.3(SDA/SDI/SDO) U504.6(SDA/SDI/SDO) U505.24(SDA/SDI) U506.7(SDI/SDA) X503.8 ; also sheet 1
SPI_INT_SCK: U501.2(SCL/SPC) U502.2(SCL/SPC) U504.4(SCL/SPC) U505.23(SCL/SCLK) U506.8(SCLK) X503.10 ; also sheet 1
VDD_3V3_SENSORS [power]: C501.P$1 C502.P$1 C503.P$1 C506.P$1 C507.P$1 C508.P$1 C511.P$1 C513.P$1 C514.P$1 U501.1(VDD_IO) U501.15(RES_P15_VDD) U501.16(VDD) U502.1(VDD_IO) U502.15(VDD) U502.16(VDD) U504.1(VDD_IO) U504.14(VDD) U505.13(VDD) U506.1(VDD) X503.1 ; also sheet 6,12
Unconnected: U501.7(INT1) U502.7(INT1) U502.8(DEN) U505.2(NC1) U505.3(NC2) U505.4(NC3) U505.5(NC4) U505.6(AUX_DA) U505.7(AUX_CL) U505.11(FSYNC) U505.14(NC5) U505.15(NC6) U505.16(NC7) U505.17(NC8) U505.19(RESV1) U505.21(RESV2) U505.22(CLKOUT) U506.4(CSB1)

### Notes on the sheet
- NOTE: place 10uF cap
  close to gyros
- Stuff option 1: L3GD20 (legacy gyro)
- Stuff option 4: onboard accel/mag
- STUFF C503 WITH 220R RESISTOR
- Switch to L3GD20H
  once available (Q3/2013)
  WARNING: DIFFERENT HW,
  SW COMPATIBLE
- Stuff option 2: L3GD20H (replacement gyro) | Stuff option 5: MPU6000
- Valid stuff option combos:
    1 + 4 + 5
    2 + 4 + 5
    3 + 5 ONLY
  
  DO NOT stuff 1 + 2 at the same time
  DO NOT stuff 3 with any of 1, 2 or 4
- Sensors
- Stuff option 3: offboard gyro/accel/mag

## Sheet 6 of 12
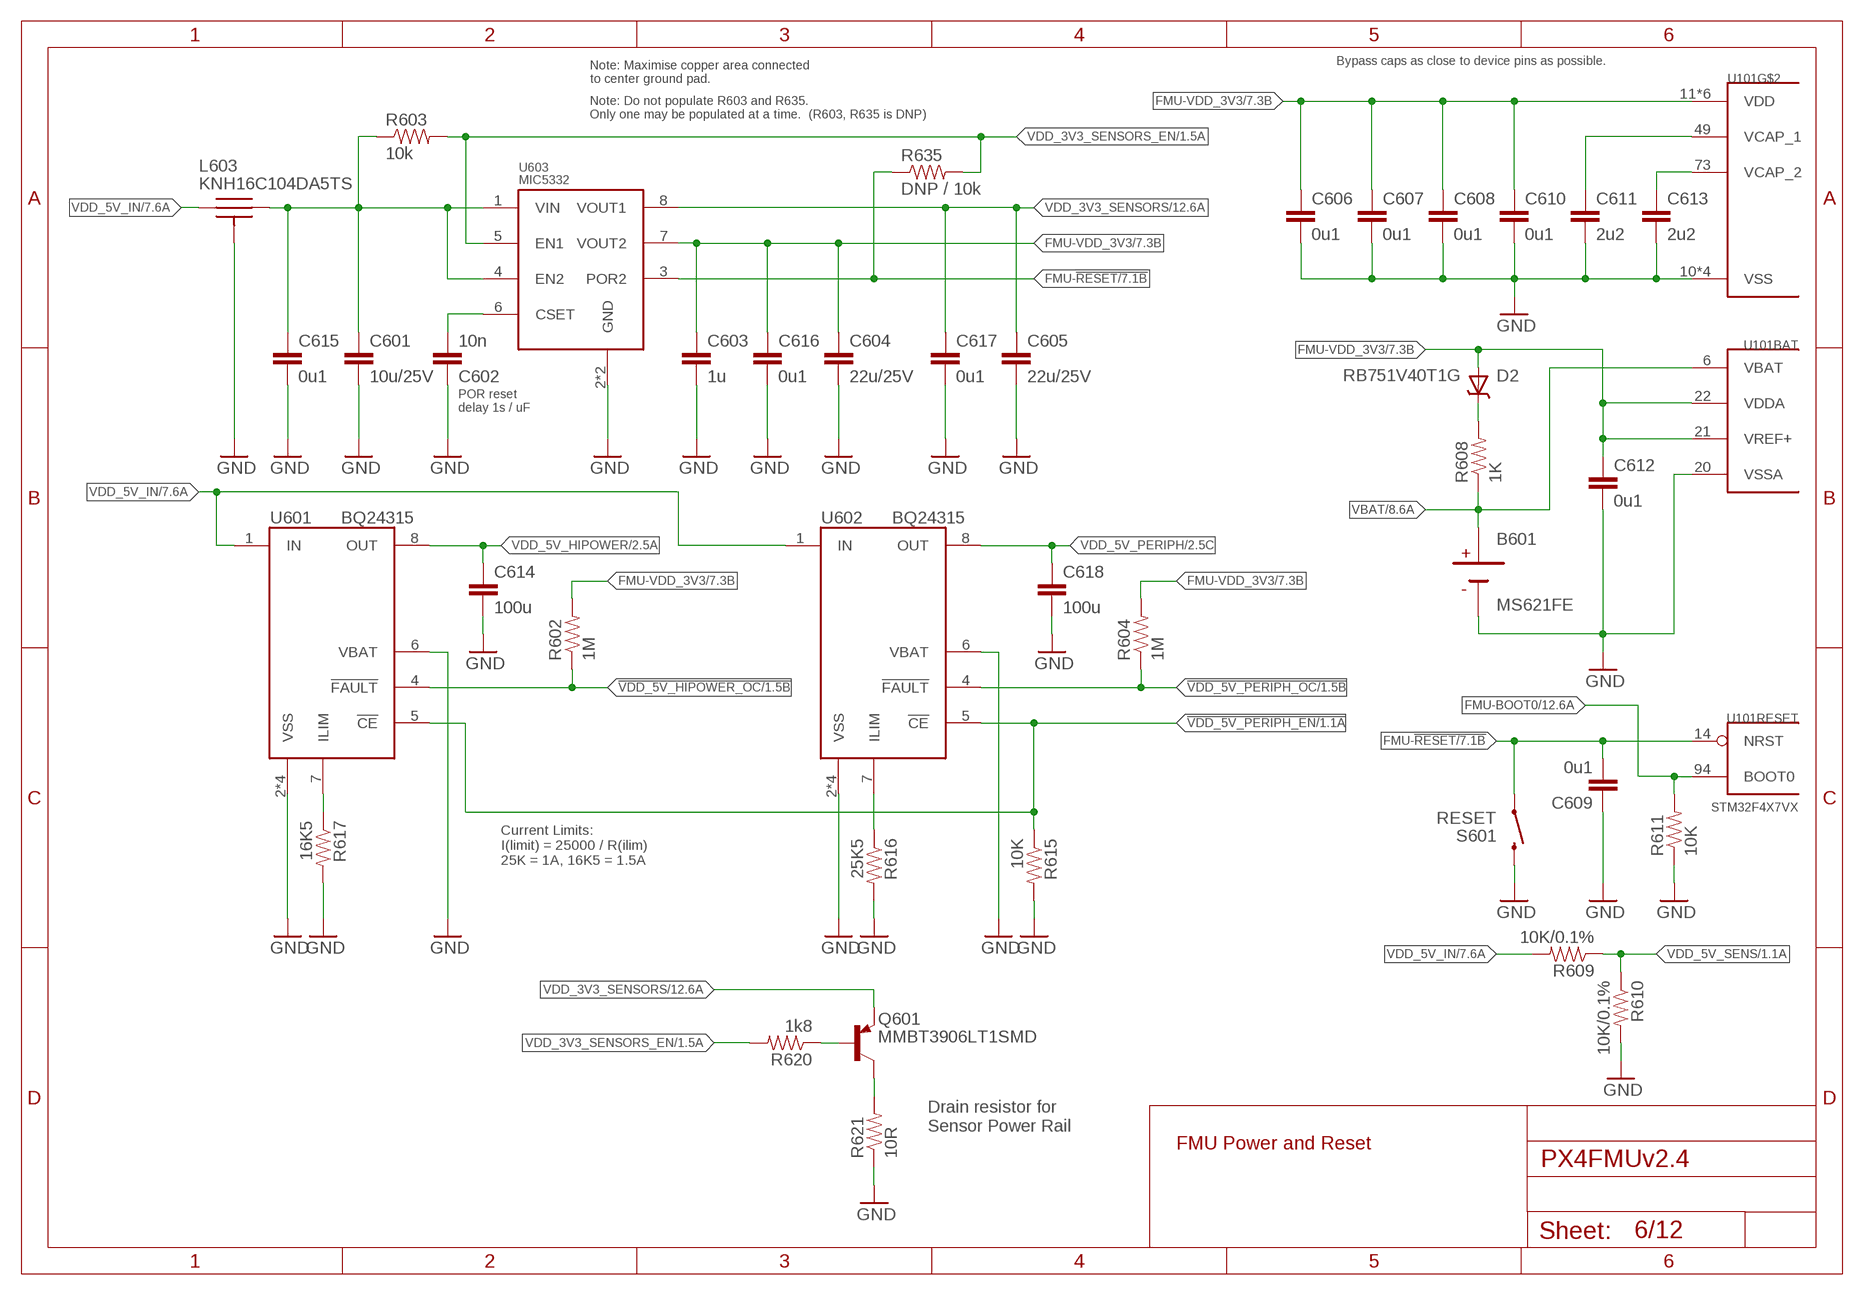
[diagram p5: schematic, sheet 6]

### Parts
B601  MS621FE  [MS621FE]
C601  10u/25V  CAP0805  [0805-CAP]
C602  10n  CAP0402  [0402-CAP]
C603  1u  CAP0603  [0603-CAP]
C604  22u/25V  CAP0805  [0805-CAP]
C605  22u/25V  CAP0805  [0805-CAP]
C606  0u1  CAP0402  [0402-CAP]
C607  0u1  CAP0402  [0402-CAP]
C608  0u1  CAP0402  [0402-CAP]
C609  0u1  CAP0402  [0402-CAP]
C610  0u1  CAP0402  [0402-CAP]
C611  2u2  CAP0603  [0603-CAP]
C612  0u1  CAP0402  [0402-CAP]
C613  2u2  CAP0603  [0603-CAP]
C614  100u  CAP1206  [1206-CAP]
C615  0u1  CAP0402  [0402-CAP]
C616  0u1  CAP0402  [0402-CAP]
C617  0u1  CAP0402  [0402-CAP]
C618  100u  CAP1206  [1206-CAP]
D2  RB751V40T1G  DIODE-SCHOTTKY_SOD323  [SOD323]
L603  KNH16C104DA5TS  [KYOCERA-KNH16-DA]
Q601  MMBT3906LT1SMD  [SOT23-BEC]
R602  1M  RESISTOR0402-RES  [0402-RES]
R603  10k  RESISTOR0402-RES  [0402-RES]
R604  1M  RESISTOR0402-RES  [0402-RES]
R608  1K  RESISTOR0402-RES  [0402-RES]
R609  10K/0.1%  RESISTOR0402-RES  [0402-RES]
R610  10K/0.1%  RESISTOR0402-RES  [0402-RES]
R611  10K  RESISTOR0402-RES  [0402-RES]
R615  10K  RESISTOR0402-RES  [0402-RES]
R616  25K5  RESISTOR0402-RES  [0402-RES]
R617  16K5  RESISTOR0402-RES  [0402-RES]
R620  1k8  RESISTOR0402-RES  [0402-RES]
R621  10R  RESISTOR0603-RES  [0603-RES]
R635  DNP / 10k  RESISTOR0402-RES  [0402-RES]
S601  RESET  SWITCH-MOMENTARY-2  [EVQP7J01K]
U601  BQ24315  [QFN8-DSG]
U602  BQ24315  [QFN8-DSG]
U603  MIC5332  [MLF-8-EPAD]

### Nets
!VDD_5V_HIPOWER_OC: R602.P$1 U601.4(!FAULT) ; also sheet 1
!VDD_5V_PERIPH_EN: R615.P$1 U601.5(!CE) U602.5(!CE) ; also sheet 1
!VDD_5V_PERIPH_OC: R604.P$1 U602.4(!FAULT) ; also sheet 1
FMU-!RESET: C609.P$2 R635.P$1 S601.A1 U101.14(RESET:NRST) U603.3(POR2) ; also sheet 7
FMU-BOOT0: R611.P$2 U101.94(RESET:BOOT0) ; also sheet 12
FMU-VDD_3V3 [power]: C603.P$1 C604.P$1 C606.P$1 C607.P$1 C608.P$1 C610.P$1 C612.P$1 C616.P$1 D2.A R602.P$2 R604.P$2 U101.11(VDD) U101.19(VDD) U101.21(BAT:VREF+) U101.22(BAT:VDDA) U101.28(VDD) U101.50(VDD) U101.75(VDD) U101.100(VDD) U603.7(VOUT2) ; also sheet 1,2,3,4,7,9,12
FMU-VDD_5V5 [power]: C601.P$1 C615.P$1 L603.P$2 R603.P$1 U603.1(VIN) U603.4(EN2)
GND [power]: B601.2(NEG) C601.P$2 C602.P$1 C603.P$2 C604.P$2 C605.P$2 C606.P$2 C607.P$2 C608.P$2 C609.P$1 C610.P$2 C611.P$2 C612.P$2 C613.P$2 C614.P$2 C615.P$2 C616.P$2 C617.P$2 C618.P$2 L603.P$3 L603.P$4 L603.P$5 R610.P$2 R611.P$1 R615.P$2 R616.P$2 R617.P$2 R621.1 S601.B3 U101.10(VSS) U101.20(BAT:VSSA) U101.27(VSS) U101.74(VSS) U101.99(VSS) U601.2(VSS) U601.6(VBAT) U601.GND(VSS) U601.P$2(VSS) U601.P$3(VSS) U602.2(VSS) U602.6(VBAT) U602.GND(VSS) U602.P$2(VSS) U602.P$3(VSS) U603.2(GND) U603.GND ; also sheet 1,2,3,4,5,7,8,9,10,11,12
N$8: C613.P$1 U101.73(VCAP_2)
N$11: C602.P$2 U603.6(CSET)
N$12: C611.P$1 U101.49(VCAP_1)
N$21: D2.C R608.P$2
N$34: R616.P$1 U602.7(ILIM)
N$80: Q601.C R621.2
N$81: Q601.B R620.P$1
N$96: R617.P$1 U601.7(ILIM)
VBAT: B601.1(POS) R608.P$1 U101.6(BAT:VBAT) ; also sheet 8
VDD_3V3_SENSORS [power]: C605.P$1 C617.P$1 Q601.E U603.8(VOUT1) ; also sheet 5,12
VDD_3V3_SENSORS_EN: R603.P$2 R620.P$2 R635.P$2 U603.5(EN1) ; also sheet 1
VDD_5V_HIPOWER [power]: C614.P$1 U601.8(OUT) ; also sheet 2
VDD_5V_IN [power]: L603.P$1 R609.P$2 U601.1(IN) U602.1(IN) ; also sheet 7,10,11,12
VDD_5V_PERIPH [power]: C618.P$1 U602.8(OUT) ; also sheet 2,4
VDD_5V_SENS: R609.P$1 R610.P$1 ; also sheet 1

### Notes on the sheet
- Bypass caps as close to device pins as possible.
- Note: Maximise copper area connected 
  to center ground pad.
- Note: Do not populate R603 and R635.  
  Only one may be populated at a time.  (R603, R635 is DNP)
- POR reset 
  delay 1s / uF
- Current Limits:
  I(limit) = 25000 / R(ilim)
  25K = 1A, 16K5 = 1.5A
- Drain resistor for 
  Sensor Power Rail
- FMU Power and Reset

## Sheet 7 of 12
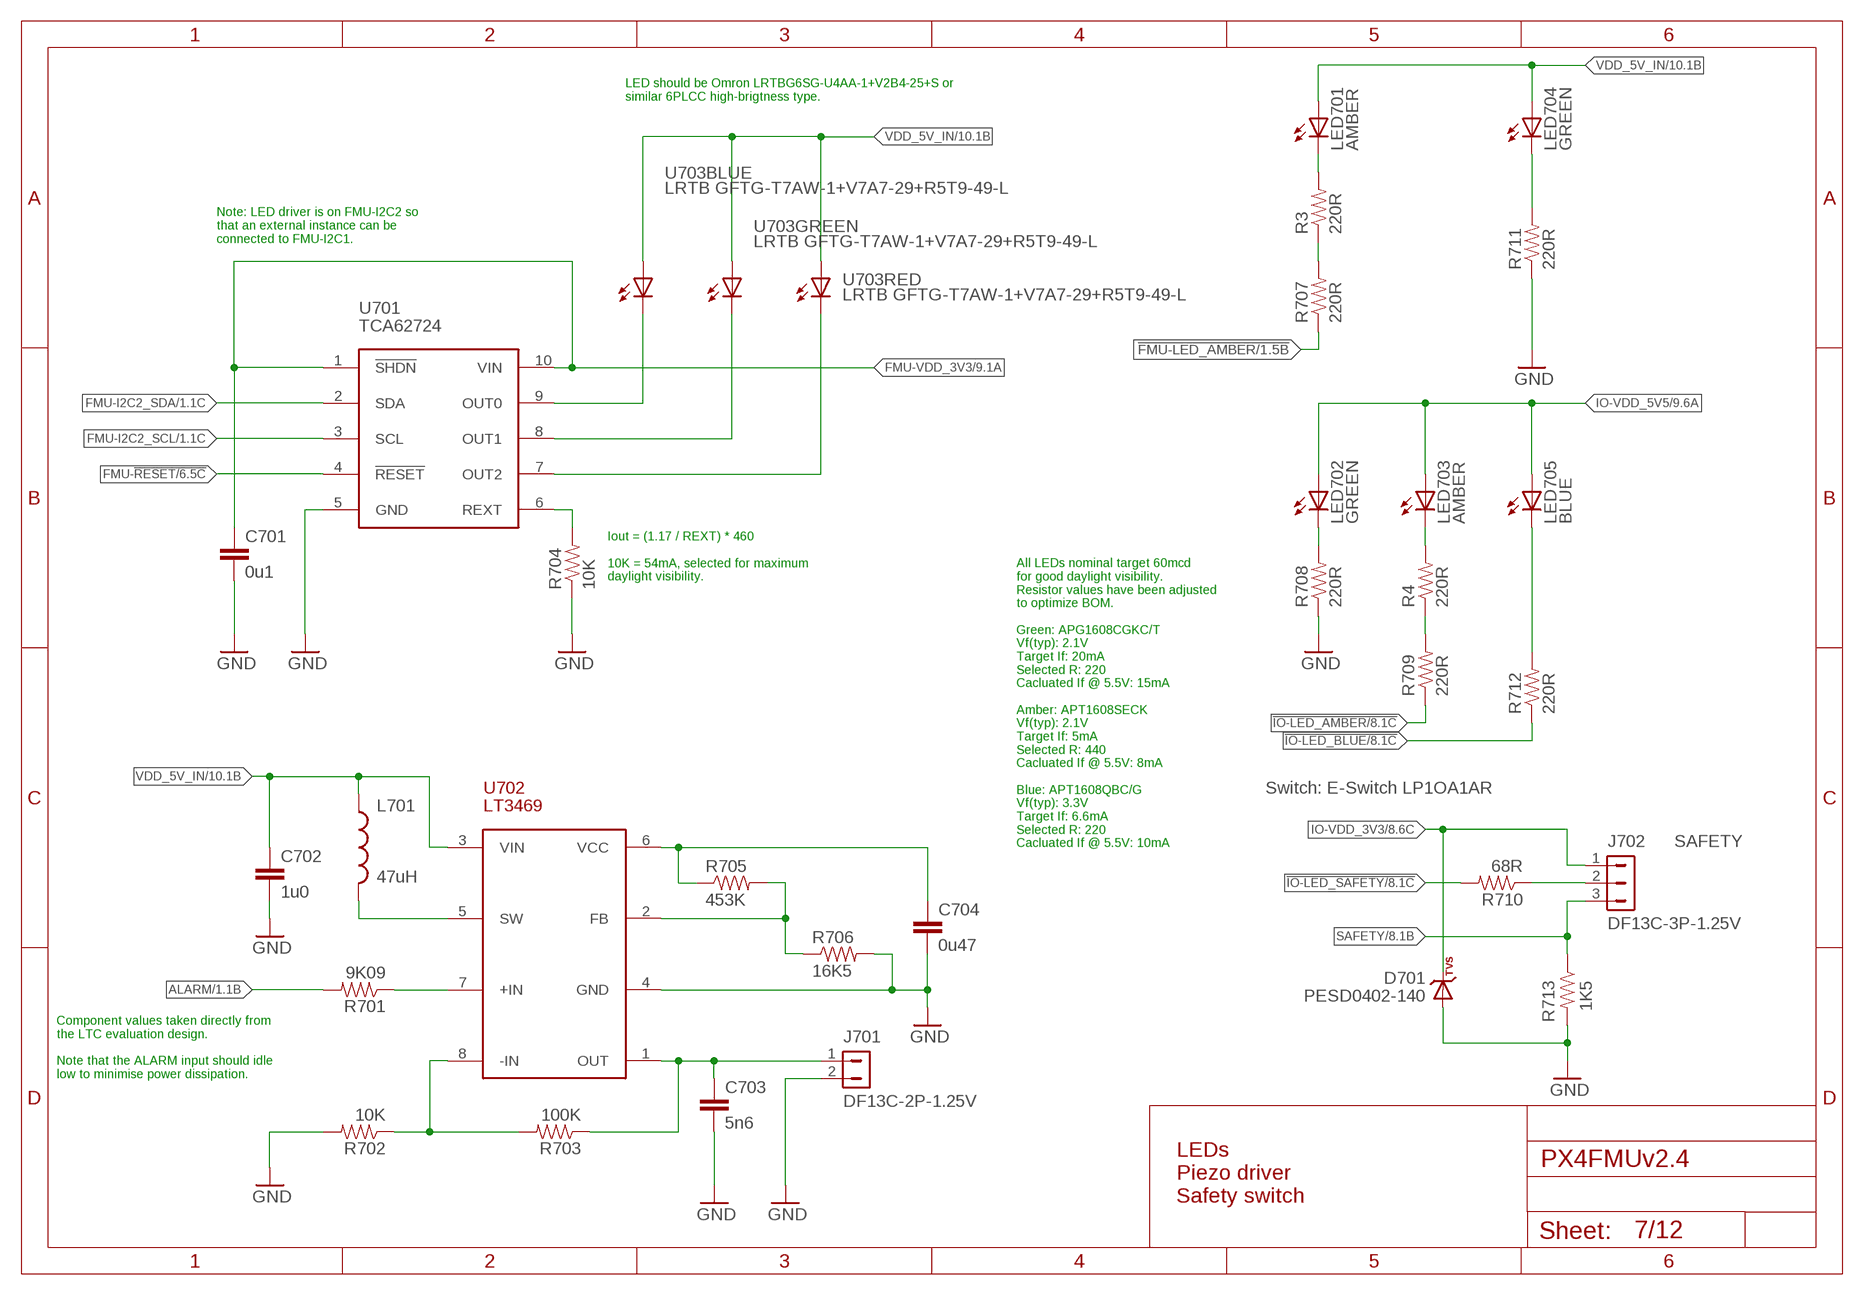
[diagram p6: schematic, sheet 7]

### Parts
C701  0u1  CAP0402  [0402-CAP]
C702  1u0  CAP0603  [0603-CAP]
C703  5n6  CAP0402  [0402-CAP]
C704  0u47  CAP0402  [0402-CAP]
D701  PESD0402-140  DIODE-TVS  [0402-TVS]
J701  DF13C-2P-1.25V  DF13-2P-1.25V  [DF13C-2P-1.25V]
J702  DF13C-3P-1.25V  DF13-3P-1.25V  [DF13C-3P-1.25V]
L701  47uH  INDUCTOR0805  [0805-IND]
LED701  AMBER  LED0603  [0603-LED]
LED702  GREEN  LED0603  [0603-LED]
LED703  AMBER  LED0603  [0603-LED]
LED704  GREEN  LED0603  [0603-LED]
LED705  BLUE  LED0603  [0603-LED]
R3  220R  RESISTOR0402-RES  [0402-RES]
R4  220R  RESISTOR0402-RES  [0402-RES]
R701  9K09  RESISTOR0402-RES  [0402-RES]
R702  10K  RESISTOR0402-RES  [0402-RES]
R703  100K  RESISTOR0402-RES  [0402-RES]
R704  10K  RESISTOR0402-RES  [0402-RES]
R705  453K  RESISTOR0402-RES  [0402-RES]
R706  16K5  RESISTOR0402-RES  [0402-RES]
R707  220R  RESISTOR0402-RES  [0402-RES]
R708  220R  RESISTOR0402-RES  [0402-RES]
R709  220R  RESISTOR0402-RES  [0402-RES]
R710  68R  RESISTOR0402-RES  [0402-RES]
R711  220R  RESISTOR0402-RES  [0402-RES]
R712  220R  RESISTOR0402-RES  [0402-RES]
R713  1K5  RESISTOR0402-RES  [0402-RES]
U701  TCA62724FMG  [SON10]
U702  LT3469  [SOT23-8]
U703  LRTB GFTG-T7AW-1+V7A7-29+R5T9-49-L  RGB-LED6-PLCC  [6-PLCC]

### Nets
!FMU-LED_AMBER: R707.P$1 ; also sheet 1
!IO-LED_AMBER: R709.P$1 ; also sheet 8
!IO-LED_BLUE: R712.P$1 ; also sheet 8
!IO-LED_SAFETY: R710.P$2 ; also sheet 8
ALARM: R701.P$2 ; also sheet 1
FMU-!RESET: U701.4(!RESET) ; also sheet 6
FMU-I2C2_SCL: U701.3(SCL) ; also sheet 1,3
FMU-I2C2_SDA: U701.2(SDA) ; also sheet 1,3
FMU-VDD_3V3 [power]: C701.P$1 U701.1(!SHDN) U701.10(VIN) ; also sheet 1,2,3,4,6,9,12
GND [power]: C701.P$2 C702.P$2 C703.P$2 C704.P$2 D701.A J701.2 R702.P$2 R704.P$1 R706.P$2 R708.P$1 R711.P$1 R713.P$2 U701.5(GND) U702.4(GND) ; also sheet 1,2,3,4,5,6,8,9,10,11,12
IO-VDD_3V3 [power]: D701.C J702.1 ; also sheet 8,9,10
IO-VDD_5V5 [power]: LED702.A LED703.A LED705.A ; also sheet 9,10
N$7: LED704.C R711.P$2
N$9: LED705.C R712.P$2
N$13: R3.P$1 R707.P$2
N$24: R705.P$2 R706.P$1 U702.2(FB)
N$25: R702.P$1 R703.P$2 U702.8(-IN)
N$26: LED701.C R3.P$2
N$27: C703.P$1 J701.1 R703.P$1 U702.1(OUT)
N$28: R701.P$1 U702.7(+IN)
N$29: LED702.C R708.P$2
N$32: L701.P$2 U702.5(SW)
N$36: C704.P$1 R705.P$1 U702.6(VCC)
N$39: R4.P$1 R709.P$2
N$40: LED703.C R4.P$2
N$57: J702.2 R710.P$1
N$95: R704.P$2 U701.6(REXT)
RGB_LED_3: U701.9(OUT0) U703.C1(BLUE:C)
RGB_LED_4: U701.8(OUT1) U703.C2(GREEN:C)
RGB_LED_14: U701.7(OUT2) U703.C3(RED:C)
SAFETY: J702.3 R713.P$1 ; also sheet 8
VDD_5V_IN [power]: C702.P$1 L701.P$1 LED701.A LED704.A U702.3(VIN) U703.A1(BLUE:A) U703.A2(GREEN:A) U703.A3(RED:A) ; also sheet 6,10,11,12

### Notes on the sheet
- LED should be Omron LRTBG6SG-U4AA-1+V2B4-25+S or 
  similar 6PLCC high-brigtness type.
- Note: LED driver is on FMU-I2C2 so
  that an external instance can be
  connected to FMU-I2C1.
- Iout = (1.17 / REXT) * 460
  
  10K = 54mA, selected for maximum
  daylight visibility.
- Switch: E-Switch LP1OA1AR
- All LEDs nominal target 60mcd
  for good daylight visibility.
  Resistor values have been adjusted
  to optimize BOM.
  
  Green: APG1608CGKC/T
  Vf(typ): 2.1V
  Target If: 20mA
  Selected R: 220
  Cacluated If @ 5.5V: 15mA
  
  Amber: APT1608SECK
  Vf(typ): 2.1V
  Target If: 5mA
  Selected R: 440
  Cacluated If @ 5.5V: 8mA
  
  Blue: APT1608QBC/G
  Vf(typ): 3.3V
  Target If: 6.6mA
  Selected R: 220
  Cacluated If @ 5.5V: 10mA
- SAFETY
- Component values taken directly from
  the LTC evaluation design.
  
  Note that the ALARM input should idle
  low to minimise power dissipation.
- LEDs
  Piezo driver
  Safety switch

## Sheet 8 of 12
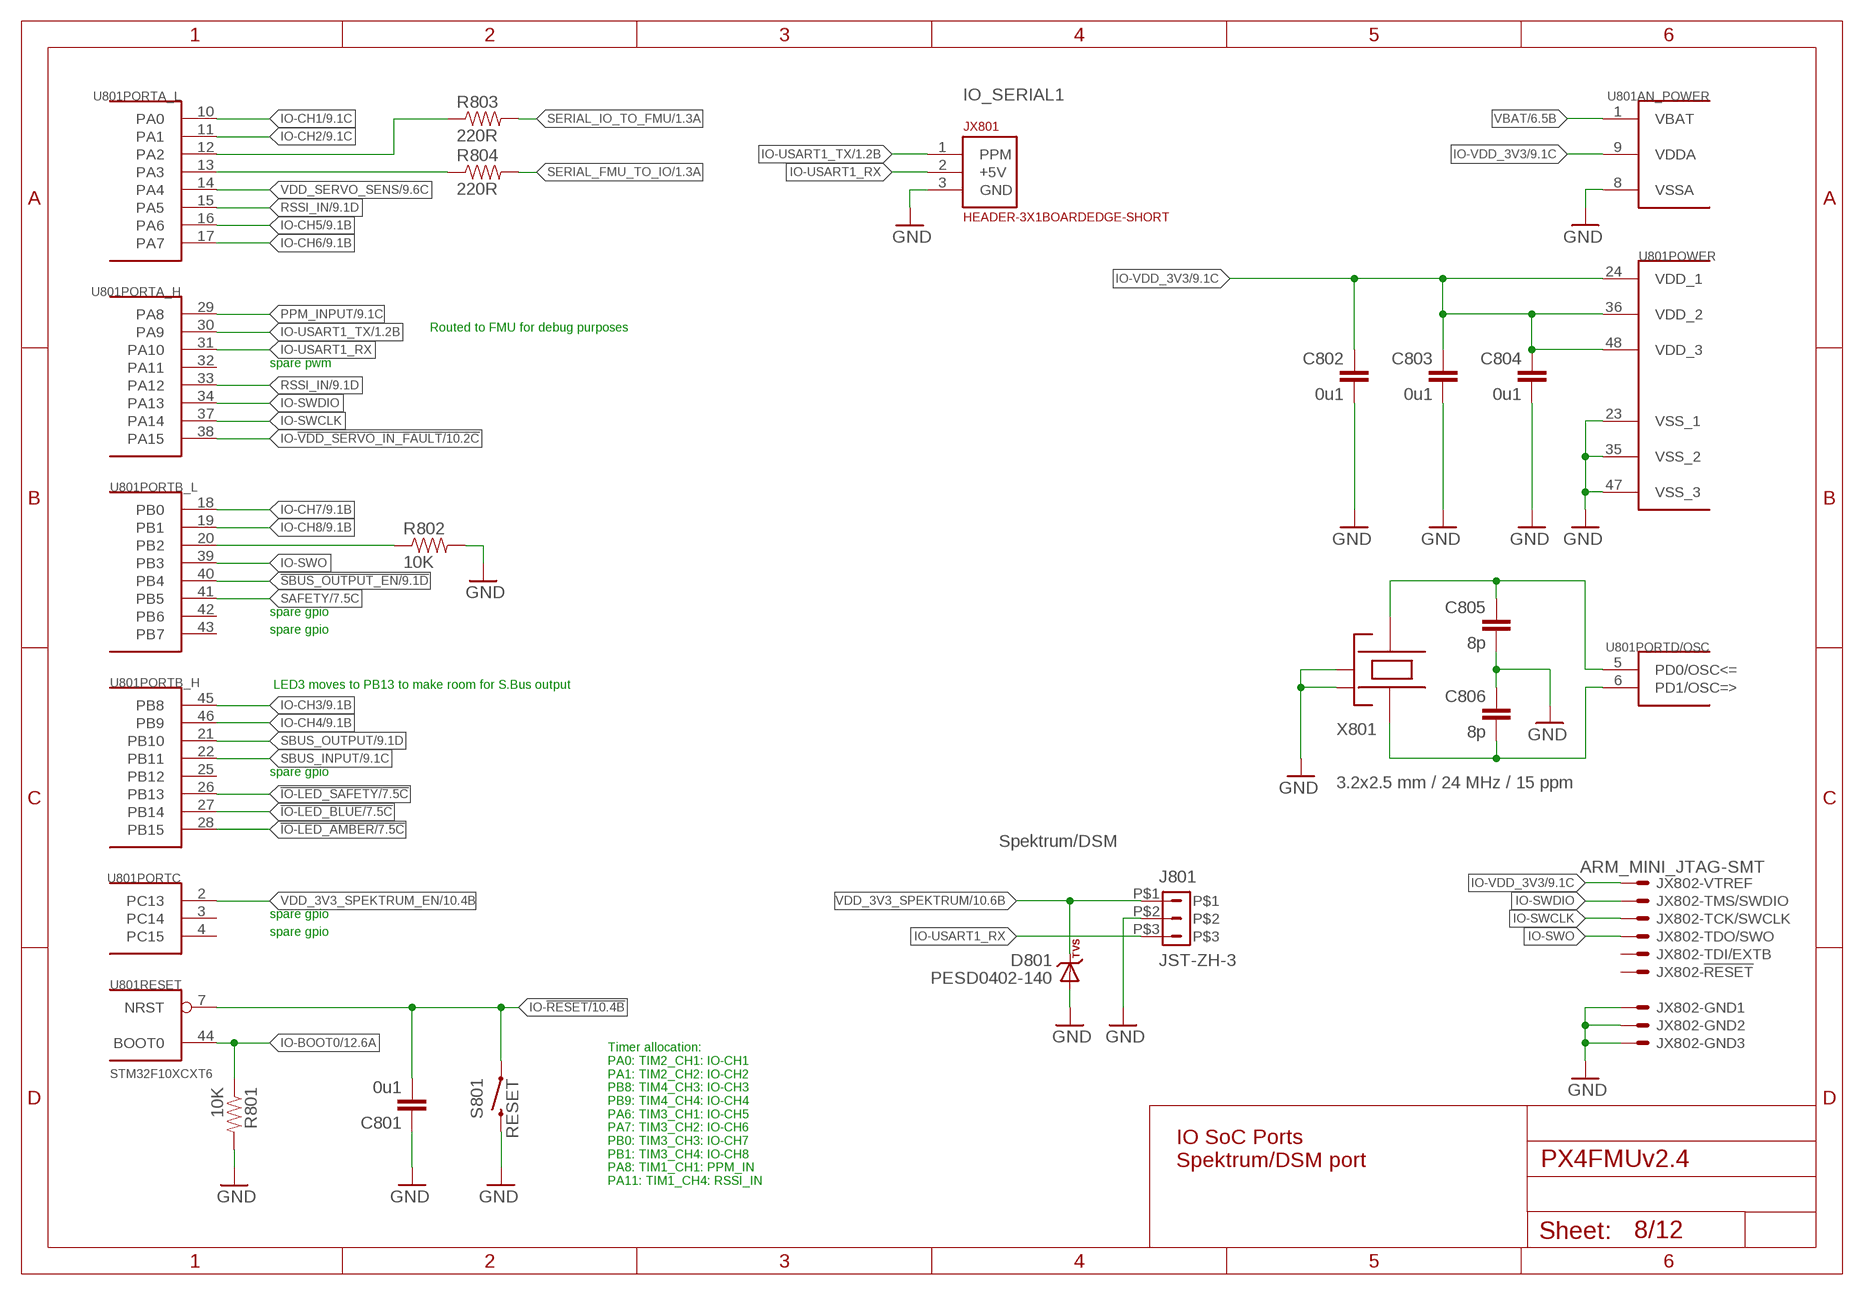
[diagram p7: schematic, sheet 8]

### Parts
C801  0u1  CAP0402  [0402-CAP]
C802  0u1  CAP0402  [0402-CAP]
C803  0u1  CAP0402  [0402-CAP]
C804  0u1  CAP0402  [0402-CAP]
C805  8p  CAP0402  [0402-CAP]
C806  8p  CAP0402  [0402-CAP]
D801  PESD0402-140  DIODE-TVS  [0402-TVS]
J801  JST-ZH-3  [JST-ZH-SMT-VERTICAL]
JX801  HEADER-3X1BOARDEDGE-SHORT  [HEADER_3X01_SMD_H_BOARD_EDGE_SHORT]
JX802  ARM_MINI_JTAG-SMT  [FTSH-105-01-XXX-DV-K]
R801  10K  RESISTOR0402-RES  [0402-RES]
R802  10K  RESISTOR0402-RES  [0402-RES]
R803  220R  RESISTOR0402-RES  [0402-RES]
R804  220R  RESISTOR0402-RES  [0402-RES]
S801  RESET  SWITCH-MOMENTARY-2  [EVQP7J01K]
U801  STM32F10XCXT6  [TQFP48]
X801  3.2x2.5 mm / 24 MHz / 15 ppm  OSCILLATOR-3.2X2.5  [OSCILLATOR-3.2X2.5]

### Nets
!IO-LED_AMBER: U801.28(PORTB_H:PB15) ; also sheet 7
!IO-LED_BLUE: U801.27(PORTB_H:PB14) ; also sheet 7
!IO-LED_SAFETY: U801.26(PORTB_H:PB13) ; also sheet 7
!SBUS_OUTPUT_EN: U801.40(PORTB_L:PB4) ; also sheet 9
GND [power]: C801.P$1 C802.P$2 C803.P$2 C804.P$2 C805.P$2 C806.P$1 D801.A J801.P$2 JX801.3(GND) JX802.3 JX802.5 JX802.9 R801.P$2 R802.P$2 S801.B3 U801.8(AN_POWER:VSSA) U801.23(POWER:VSS_1) U801.35(POWER:VSS_2) U801.47(POWER:VSS_3) X801.2(NC_2) X801.4(NC_4) ; also sheet 1,2,3,4,5,6,7,9,10,11,12
IO-!RESET: C801.P$2 S801.A1 U801.7(RESET:NRST) ; also sheet 10
IO-!VDD_SERVO_IN_FAULT: U801.38(PORTA_H:PA15) ; also sheet 10
IO-BOOT0: R801.P$1 U801.44(RESET:BOOT0) ; also sheet 12
IO-BOOT1: R802.P$1 U801.20(PORTB_L:PB2)
IO-CH1: U801.10(PORTA_L:PA0) ; also sheet 9
IO-CH2: U801.11(PORTA_L:PA1) ; also sheet 9
IO-CH3: U801.45(PORTB_H:PB8) ; also sheet 9
IO-CH4: U801.46(PORTB_H:PB9) ; also sheet 9
IO-CH5: U801.16(PORTA_L:PA6) ; also sheet 9
IO-CH6: U801.17(PORTA_L:PA7) ; also sheet 9
IO-CH7: U801.18(PORTB_L:PB0) ; also sheet 9
IO-CH8: U801.19(PORTB_L:PB1) ; also sheet 9
IO-SWCLK: JX802.4 U801.37(PORTA_H:PA14)
IO-SWDIO: JX802.2 U801.34(PORTA_H:PA13)
IO-SWO: JX802.6 U801.39(PORTB_L:PB3)
IO-USART1_RX: J801.P$3 JX801.2(+5V) U801.31(PORTA_H:PA10)
IO-USART1_TX: JX801.1(PPM) U801.30(PORTA_H:PA9) ; also sheet 1
IO-VDD_3V3 [power]: C802.P$1 C803.P$1 C804.P$1 JX802.1 U801.9(AN_POWER:VDDA) U801.24(POWER:VDD_1) U801.36(POWER:VDD_2) U801.48(POWER:VDD_3) ; also sheet 7,9,10
N$15: R803.P$1 U801.12(PORTA_L:PA2)
N$16: R804.P$1 U801.13(PORTA_L:PA3)
N$18: C806.P$2 U801.6(PORTD/OSC:PD1/OSC=>) X801.1
N$22: C805.P$1 U801.5(PORTD/OSC:PD0/OSC<=) X801.3
PPM_INPUT: U801.29(PORTA_H:PA8) ; also sheet 9
RSSI_IN: U801.15(PORTA_L:PA5) U801.33(PORTA_H:PA12) ; also sheet 9
SAFETY: U801.41(PORTB_L:PB5) ; also sheet 7
SBUS_INPUT: U801.22(PORTB_H:PB11) ; also sheet 9
SBUS_OUTPUT: U801.21(PORTB_H:PB10) ; also sheet 9
SERIAL_FMU_TO_IO: R804.P$2 ; also sheet 1
SERIAL_IO_TO_FMU: R803.P$2 ; also sheet 1
VBAT: U801.1(AN_POWER:VBAT) ; also sheet 6
VDD_3V3_SPEKTRUM [power]: D801.C J801.P$1 ; also sheet 10
VDD_3V3_SPEKTRUM_EN: U801.2(PORTC:PC13) ; also sheet 10
VDD_SERVO_SENS: U801.14(PORTA_L:PA4) ; also sheet 9
Unconnected: JX802.8 JX802.10 U801.3(PORTC:PC14) U801.4(PORTC:PC15) U801.25(PORTB_H:PB12) U801.32(PORTA_H:PA11) U801.42(PORTB_L:PB6) U801.43(PORTB_L:PB7)

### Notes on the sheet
- IO_SERIAL1
- Routed to FMU for debug purposes
- spare pwm
- spare gpio
- spare gpio
- LED3 moves to PB13 to make room for S.Bus output
- spare gpio
- Spektrum/DSM
- spare gpio
- spare gpio
- IO SoC Ports
  Spektrum/DSM port
- Timer allocation:
  PA0: TIM2_CH1: IO-CH1
  PA1: TIM2_CH2: IO-CH2
  PB8: TIM4_CH3: IO-CH3
  PB9: TIM4_CH4: IO-CH4
  PA6: TIM3_CH1: IO-CH5
  PA7: TIM3_CH2: IO-CH6
  PB0: TIM3_CH3: IO-CH7
  PB1: TIM3_CH4: IO-CH8
  PA8: TIM1_CH1: PPM_IN
  PA11: TIM1_CH4: RSSI_IN

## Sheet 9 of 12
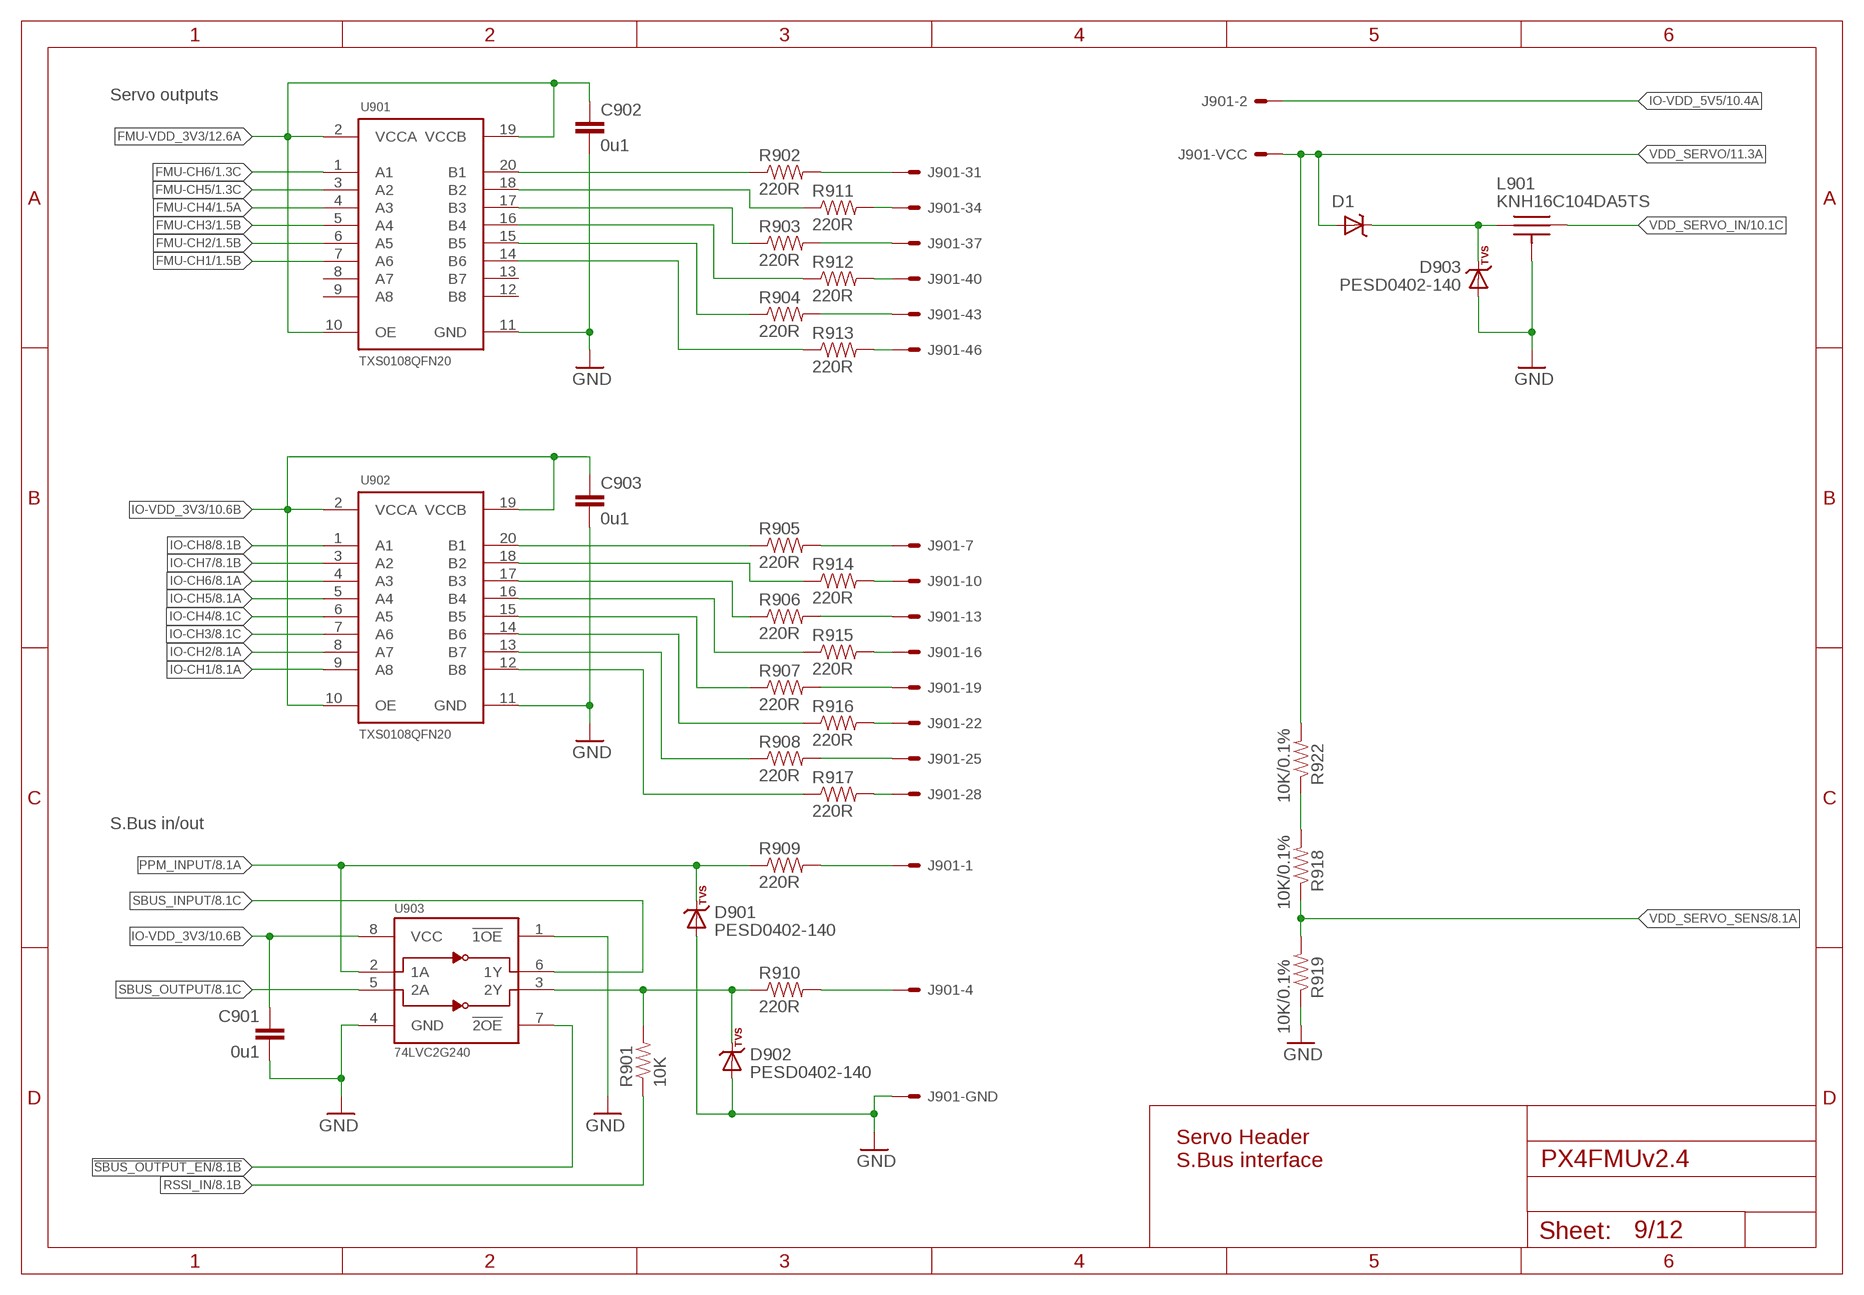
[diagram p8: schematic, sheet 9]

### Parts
C901  0u1  CAP0402  [0402-CAP]
C902  0u1  CAP0402  [0402-CAP]
C903  0u1  CAP0402  [0402-CAP]
D1  MSS1P4-M3  DIODE-SCHOTTKY_MSMP  [MICROSMP]
D901  PESD0402-140  DIODE-TVS  [0402-TVS]
D902  PESD0402-140  DIODE-TVS  [0402-TVS]
D903  PESD0402-140  DIODE-TVS  [0402-TVS]
J901  HEADER-3X163X16RA  [3X16RA]
L901  KNH16C104DA5TS  [KYOCERA-KNH16-DA]
R901  10K  RESISTOR0402-RES  [0402-RES]
R902  220R  RESISTOR0402-RES  [0402-RES]
R903  220R  RESISTOR0402-RES  [0402-RES]
R904  220R  RESISTOR0402-RES  [0402-RES]
R905  220R  RESISTOR0402-RES  [0402-RES]
R906  220R  RESISTOR0402-RES  [0402-RES]
R907  220R  RESISTOR0402-RES  [0402-RES]
R908  220R  RESISTOR0402-RES  [0402-RES]
R909  220R  RESISTOR0402-RES  [0402-RES]
R910  220R  RESISTOR0402-RES  [0402-RES]
R911  220R  RESISTOR0402-RES  [0402-RES]
R912  220R  RESISTOR0402-RES  [0402-RES]
R913  220R  RESISTOR0402-RES  [0402-RES]
R914  220R  RESISTOR0402-RES  [0402-RES]
R915  220R  RESISTOR0402-RES  [0402-RES]
R916  220R  RESISTOR0402-RES  [0402-RES]
R917  220R  RESISTOR0402-RES  [0402-RES]
R918  10K/0.1%  RESISTOR0402-RES  [0402-RES]
R919  10K/0.1%  RESISTOR0402-RES  [0402-RES]
R922  10K/0.1%  RESISTOR0402-RES  [0402-RES]
U901  TXS0108QFN20  [QFN20-RGY]
U902  TXS0108QFN20  [QFN20-RGY]
U903  74LVC2G240  74LVC2G240-TSSOP-8  [TSSOP8_SOT505-2]

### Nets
!SBUS_OUTPUT_EN: U903.7(!2OE) ; also sheet 8
FMU-CH1: U901.7(A6) ; also sheet 1
FMU-CH1-PROT: J901.46 R913.P$2
FMU-CH2: U901.6(A5) ; also sheet 1
FMU-CH3: U901.5(A4) ; also sheet 1
FMU-CH4: U901.4(A3) ; also sheet 1
FMU-CH5: U901.3(A2) ; also sheet 1
FMU-CH6: U901.1(A1) ; also sheet 1
FMU-CH6-PROT: J901.31 R902.P$2
FMU-VDD_3V3 [power]: C902.P$1 U901.2(VCCA) U901.10(OE) U901.19(VCCB) ; also sheet 1,2,3,4,6,7,12
GND [power]: C901.P$2 C902.P$2 C903.P$2 D901.A D902.A D903.A J901.3 J901.6 J901.9 J901.12 J901.15 J901.18 J901.21 J901.24 J901.27 J901.30 J901.33 J901.36 J901.39 J901.42 J901.45 J901.48 L901.P$3 L901.P$4 L901.P$5 R919.P$1 U901.11(GND) U902.11(GND) U903.1(!1OE) U903.4(GND) ; also sheet 1,2,3,4,5,6,7,8,10,11,12
IO-CH1: U902.9(A8) ; also sheet 8
IO-CH1-PROT: J901.28 R917.P$2
IO-CH2: U902.8(A7) ; also sheet 8
IO-CH3: U902.7(A6) ; also sheet 8
IO-CH4: U902.6(A5) ; also sheet 8
IO-CH5: U902.5(A4) ; also sheet 8
IO-CH6: U902.4(A3) ; also sheet 8
IO-CH7: U902.3(A2) ; also sheet 8
IO-CH8: U902.1(A1) ; also sheet 8
IO-CH8-PROT: J901.7 R905.P$2
IO-VDD_3V3 [power]: C901.P$1 C903.P$1 U902.2(VCCA) U902.10(OE) U902.19(VCCB) U903.8(VCC) ; also sheet 7,8,10
IO-VDD_5V5 [power]: J901.2 ; also sheet 7,10
N$3: R918.P$2 R922.P$1
N$31: J901.10 R914.P$2
N$38: D902.C R901.P$2 R910.P$1 U903.3(2Y)
N$43: R905.P$1 U902.20(B1)
N$44: R914.P$1 U902.18(B2)
N$45: R906.P$1 U902.17(B3)
N$49: R915.P$1 U902.16(B4)
N$53: R907.P$1 U902.15(B5)
N$58: R916.P$1 U902.14(B6)
N$59: R908.P$1 U902.13(B7)
N$60: R917.P$1 U902.12(B8)
N$61: R902.P$1 U901.20(B1)
N$62: R911.P$1 U901.18(B2)
N$63: R903.P$1 U901.17(B3)
N$64: R912.P$1 U901.16(B4)
N$65: R904.P$1 U901.15(B5)
N$66: R913.P$1 U901.14(B6)
N$68: J901.34 R911.P$2
N$71: J901.13 R906.P$2
N$72: J901.16 R915.P$2
N$73: J901.19 R907.P$2
N$74: J901.22 R916.P$2
N$75: J901.25 R908.P$2
N$77: J901.37 R903.P$2
N$78: J901.40 R912.P$2
N$79: J901.43 R904.P$2
N$99: J901.4 R910.P$2
N$110 [power]: D1.CATHODE(C) D903.C L901.P$1
PPM-SBUS-PROT: J901.1 R909.P$2
PPM_INPUT: D901.C R909.P$1 U903.2(1A) ; also sheet 8
RSSI_IN: R901.P$1 ; also sheet 8
SBUS_INPUT: U903.6(1Y) ; also sheet 8
SBUS_OUTPUT: U903.5(2A) ; also sheet 8
VDD_SERVO [power]: D1.ANODE(A) J901.5 J901.8 J901.11 J901.14 J901.17 J901.20 J901.23 J901.26 J901.29 J901.32 J901.35 J901.38 J901.41 J901.44 J901.47 R922.P$2 ; also sheet 11,12
VDD_SERVO_IN [power]: L901.P$2 ; also sheet 10
VDD_SERVO_SENS: R918.P$1 R919.P$2 ; also sheet 8
Unconnected: U901.8(A7) U901.9(A8) U901.12(B8) U901.13(B7)

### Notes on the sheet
- Servo outputs
- S.Bus in/out
- Servo Header
  S.Bus interface

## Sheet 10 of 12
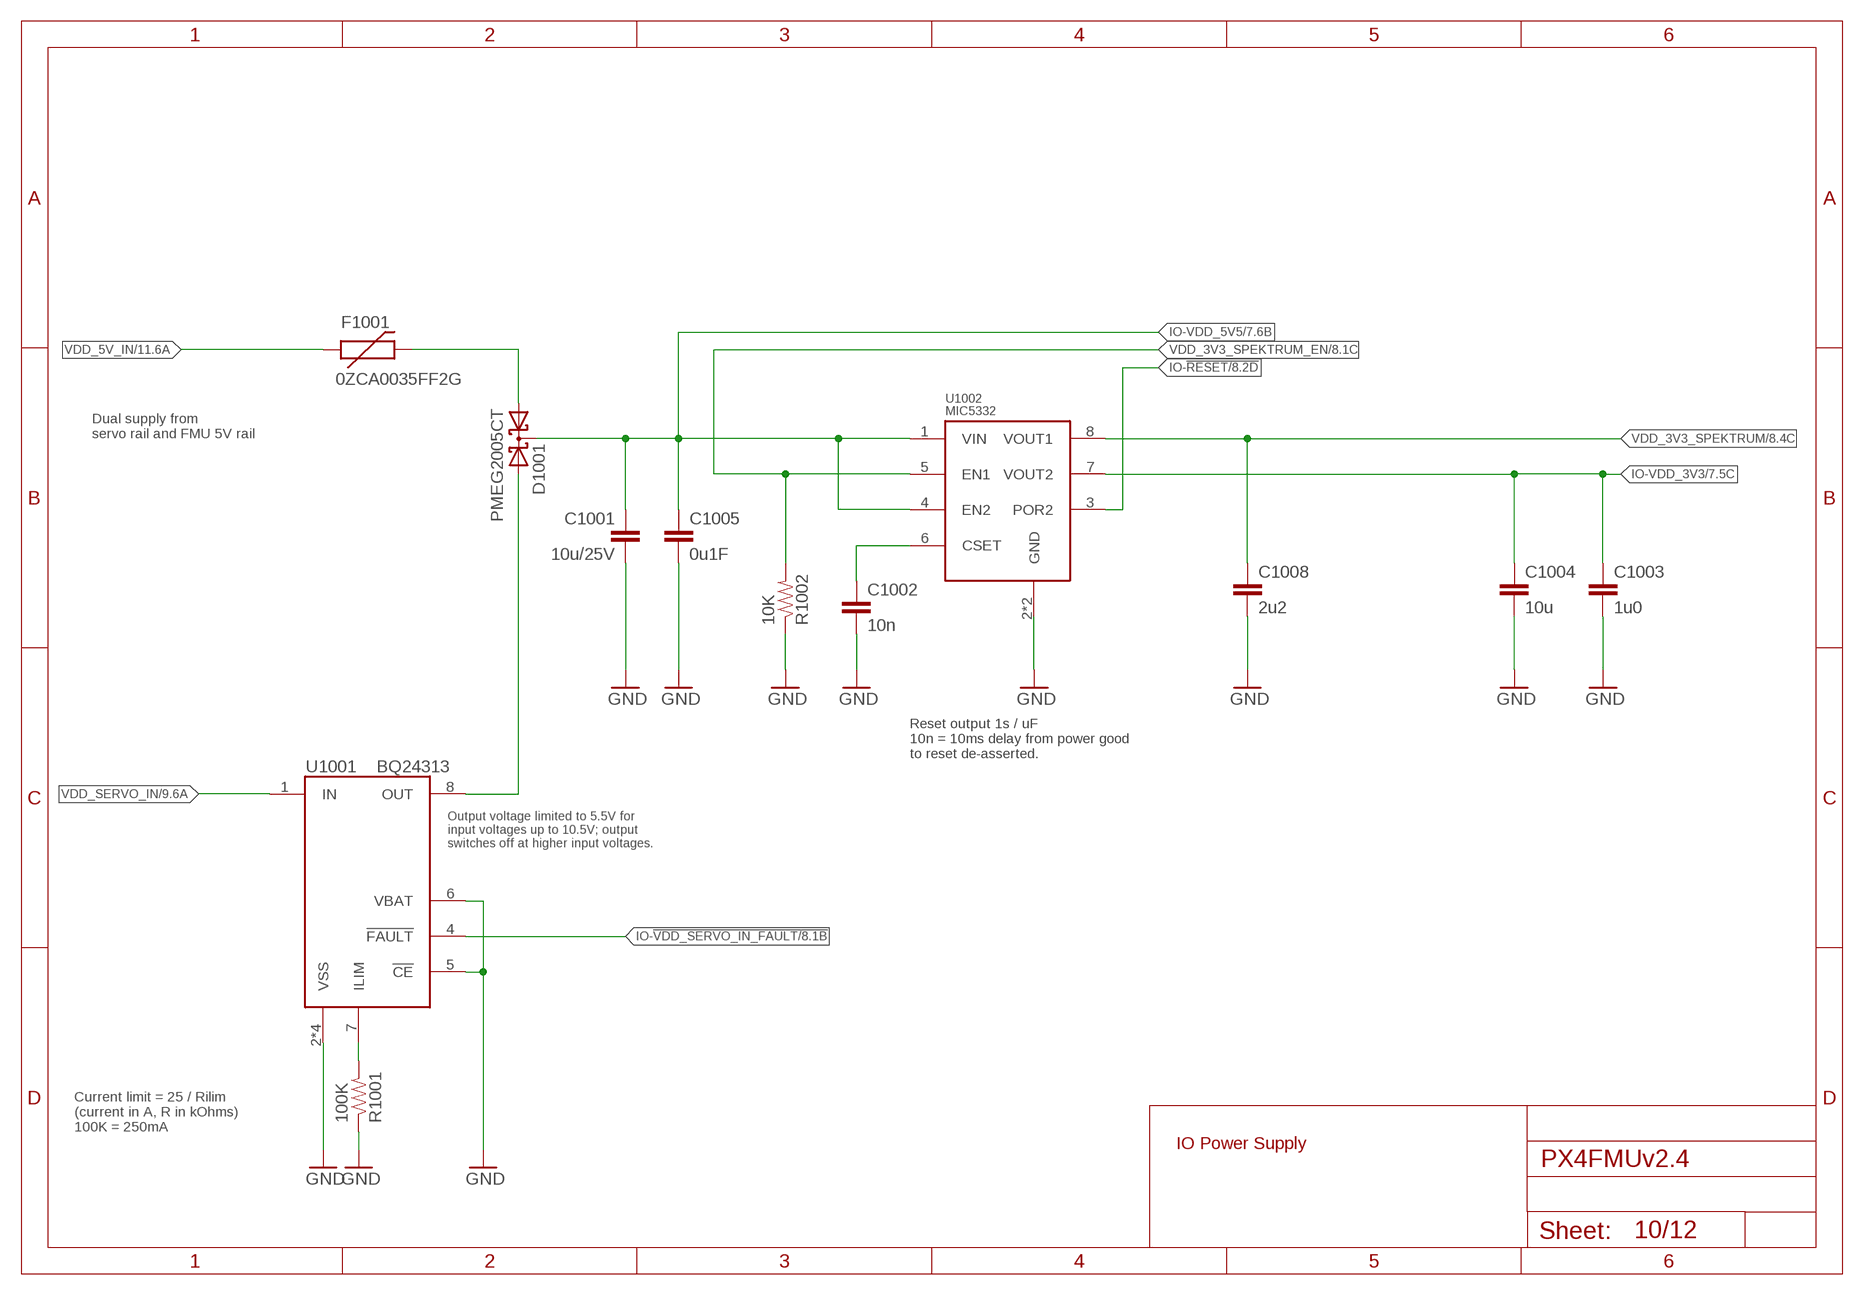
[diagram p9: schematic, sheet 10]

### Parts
C1001  10u/25V  CAP0805  [0805-CAP]
C1002  10n  CAP0402  [0402-CAP]
C1003  1u0  CAP0603  [0603-CAP]
C1004  10u  CAP0603  [0603-CAP]
C1005  0u1F  CAP0402  [0402-CAP]
C1008  2u2  CAP0402  [0402-CAP]
D1001  PMEG2005CT  [SOT23-3]
F1001  0ZCA0035FF2G  PTCSMD  [PTC-1206]
R1001  100K  RESISTOR0402-RES  [0402-RES]
R1002  10K  RESISTOR0402-RES  [0402-RES]
U1001  BQ24313  [QFN8-DSG]
U1002  MIC5332  [MLF-8-EPAD]

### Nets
GND [power]: C1001.P$2 C1002.P$2 C1003.P$2 C1004.P$2 C1005.P$2 C1008.P$2 R1001.P$1 R1002.P$1 U1001.2(VSS) U1001.5(!CE) U1001.6(VBAT) U1001.GND(VSS) U1001.P$2(VSS) U1001.P$3(VSS) U1002.2(GND) U1002.GND ; also sheet 1,2,3,4,5,6,7,8,9,11,12
IO-!RESET: U1002.3(POR2) ; also sheet 8
IO-!VDD_SERVO_IN_FAULT: U1001.4(!FAULT) ; also sheet 8
IO-VDD_3V3 [power]: C1003.P$1 C1004.P$1 U1002.7(VOUT2) ; also sheet 7,8,9
IO-VDD_5V5 [power]: C1001.P$1 C1005.P$1 D1001.3(CC) U1002.1(VIN) U1002.4(EN2) ; also sheet 7,9
N$4 [power]: D1001.2(A2) U1001.8(OUT)
N$20: R1001.P$2 U1001.7(ILIM)
N$46: D1001.1(A1) F1001.2
N$104: C1002.P$1 U1002.6(CSET)
VDD_3V3_SPEKTRUM [power]: C1008.P$1 U1002.8(VOUT1) ; also sheet 8
VDD_3V3_SPEKTRUM_EN: R1002.P$2 U1002.5(EN1) ; also sheet 8
VDD_5V_IN [power]: F1001.1 ; also sheet 6,7,11,12
VDD_SERVO_IN [power]: U1001.1(IN) ; also sheet 9

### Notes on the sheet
- Dual supply from
  servo rail and FMU 5V rail
- Reset output 1s / uF
  10n = 10ms delay from power good
  to reset de-asserted.
- Output voltage limited to 5.5V for
  input voltages up to 10.5V; output
  switches off at higher input voltages.
- Current limit = 25 / Rilim
  (current in A, R in kOhms)
  100K = 250mA
- IO Power Supply

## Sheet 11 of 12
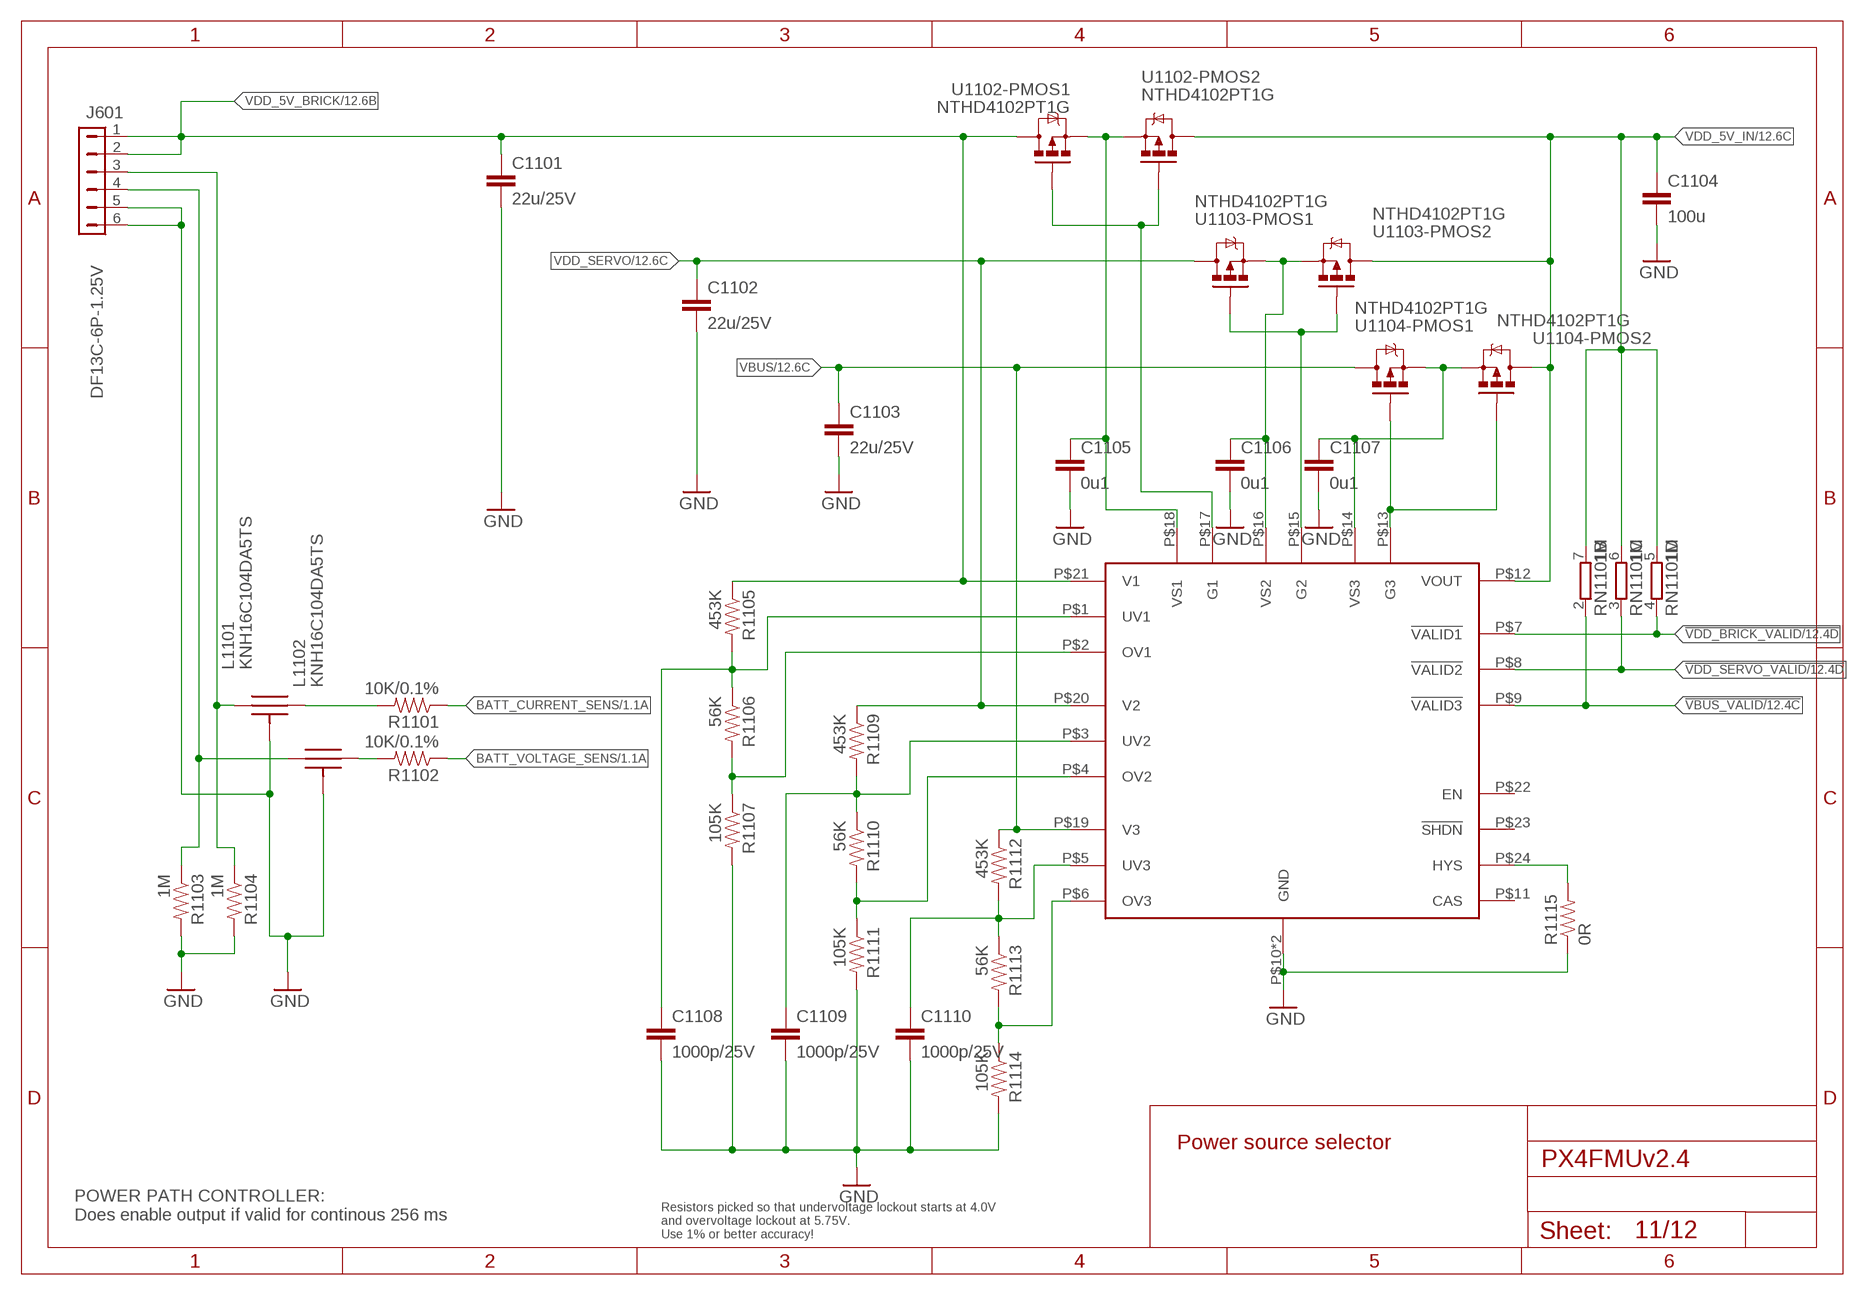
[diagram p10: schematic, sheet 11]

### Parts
C1101  22u/25V  CAP0805  [0805-CAP]
C1102  22u/25V  CAP0805  [0805-CAP]
C1103  22u/25V  CAP0805  [0805-CAP]
C1104  100u  CAP1206  [1206-CAP]
C1105  0u1  CAP0402  [0402-CAP]
C1106  0u1  CAP0402  [0402-CAP]
C1107  0u1  CAP0402  [0402-CAP]
C1108  1000p/25V  CAP0402  [0402-CAP]
C1109  1000p/25V  CAP0402  [0402-CAP]
C1110  1000p/25V  CAP0402  [0402-CAP]
J601  DF13C-6P-1.25V  DF13-6P-1.25V  [DF13C-6P-1.25V]
L1101  KNH16C104DA5TS  [KYOCERA-KNH16-DA]
L1102  KNH16C104DA5TS  [KYOCERA-KNH16-DA]
R1101  10K/0.1%  RESISTOR0402-RES  [0402-RES]
R1102  10K/0.1%  RESISTOR0402-RES  [0402-RES]
R1103  1M  RESISTOR0402-RES  [0402-RES]
R1104  1M  RESISTOR0402-RES  [0402-RES]
R1105  453K  RESISTOR0402-RES  [0402-RES]
R1106  56K  RESISTOR0402-RES  [0402-RES]
R1107  105K  RESISTOR0402-RES  [0402-RES]
R1109  453K  RESISTOR0402-RES  [0402-RES]
R1110  56K  RESISTOR0402-RES  [0402-RES]
R1111  105K  RESISTOR0402-RES  [0402-RES]
R1112  453K  RESISTOR0402-RES  [0402-RES]
R1113  56K  RESISTOR0402-RES  [0402-RES]
R1114  105K  RESISTOR0402-RES  [0402-RES]
R1115  0R  RESISTOR0402-RES  [0402-RES]
RN1101  1M  4R-NEXB28V  [EXB28V]
U1101  LTC4417  LTC4117  [MO-220]
U1102  NTHD4102PT1G  MOSFET-DUAL-PCHANNEL-CHIPFET  [1206-8]
U1103  NTHD4102PT1G  MOSFET-DUAL-PCHANNEL-CHIPFET  [1206-8]
U1104  NTHD4102PT1G  MOSFET-DUAL-PCHANNEL-CHIPFET  [1206-8]

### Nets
!VBUS_VALID: RN1101.2 U1101.P$9(!VALID3) ; also sheet 1,12
!VDD_BRICK_VALID: RN1101.4 U1101.P$7(!VALID1) ; also sheet 1,12
!VDD_SERVO_VALID: RN1101.3 U1101.P$8(!VALID2) ; also sheet 1,12
BATT_CURRENT_SENS: R1101.P$1 ; also sheet 1
BATT_CURRENT_SENS_PROT: J601.3 L1101.P$1 R1104.P$1
BATT_VOLTAGE_SENS: R1102.P$1 ; also sheet 1
BATT_VOLTAGE_SENS_PROT: J601.4 L1102.P$1 R1103.P$1
GND [power]: C1101.P$2 C1102.P$2 C1103.P$2 C1104.P$2 C1105.P$2 C1106.P$2 C1107.P$2 C1108.P$2 C1109.P$2 C1110.P$2 J601.5 J601.6 L1101.P$3 L1101.P$4 L1101.P$5 L1102.P$3 L1102.P$4 L1102.P$5 R1103.P$2 R1104.P$2 R1107.P$2 R1111.P$2 R1114.P$2 R1115.P$1 U1101.P$10(GND) U1101.P$25(GND) ; also sheet 1,2,3,4,5,6,7,8,9,10,12
N$47: C1108.P$1 R1105.P$2 R1106.P$1 U1101.P$1(UV1)
N$54: R1106.P$2 R1107.P$1 U1101.P$2(OV1)
N$55: C1109.P$1 R1109.P$2 R1110.P$1 U1101.P$3(UV2)
N$56: R1110.P$2 R1111.P$1 U1101.P$4(OV2)
N$67: R1113.P$2 R1114.P$1 U1101.P$6(OV3)
N$69: C1110.P$1 R1112.P$2 R1113.P$1 U1101.P$5(UV3)
N$97 [power]: C1105.P$1 U1101.P$18(VS1) U1102.P$1(-PMOS1:S) U1102.P$3(-PMOS2:S)
N$102: L1102.P$2 R1102.P$2
N$103: L1101.P$2 R1101.P$2
N$105: R1115.P$2 U1101.P$24(HYS)
N$106 [power]: C1106.P$1 U1101.P$16(VS2) U1103.P$1(-PMOS1:S) U1103.P$3(-PMOS2:S)
N$107 [power]: C1107.P$1 U1101.P$14(VS3) U1104.P$1(-PMOS1:S) U1104.P$3(-PMOS2:S)
N$109: U1101.P$13(G3) U1104.P$2(-PMOS1:G) U1104.P$4(-PMOS2:G)
N$113: U1101.P$15(G2) U1103.P$2(-PMOS1:G) U1103.P$4(-PMOS2:G)
N$115: U1101.P$17(G1) U1102.P$2(-PMOS1:G) U1102.P$4(-PMOS2:G)
VBUS [power]: C1103.P$1 R1112.P$1 U1101.P$19(V3) U1104.P$7(-PMOS1:D) U1104.P$8(-PMOS1:D) ; also sheet 1,3,12
VDD_5V_BRICK [power]: C1101.P$1 J601.1 J601.2 R1105.P$1 U1101.P$21(V1) U1102.P$7(-PMOS1:D) U1102.P$8(-PMOS1:D) ; also sheet 12
VDD_5V_IN [power]: C1104.P$1 RN1101.5 RN1101.6 RN1101.7 U1101.P$12(VOUT) U1102.P$5(-PMOS2:D) U1102.P$6(-PMOS2:D) U1103.P$5(-PMOS2:D) U1103.P$6(-PMOS2:D) U1104.P$5(-PMOS2:D) U1104.P$6(-PMOS2:D) ; also sheet 6,7,10,12
VDD_SERVO [power]: C1102.P$1 R1109.P$1 U1101.P$20(V2) U1103.P$7(-PMOS1:D) U1103.P$8(-PMOS1:D) ; also sheet 9,12
Unconnected: RN1101.1 RN1101.8 U1101.P$11(CAS) U1101.P$22(EN) U1101.P$23(!SHDN)

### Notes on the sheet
- Power source selector
- POWER PATH CONTROLLER:
  Does enable output if valid for continous 256 ms
- Resistors picked so that undervoltage lockout starts at 4.0V
  and overvoltage lockout at 5.75V.
  Use 1% or better accuracy!

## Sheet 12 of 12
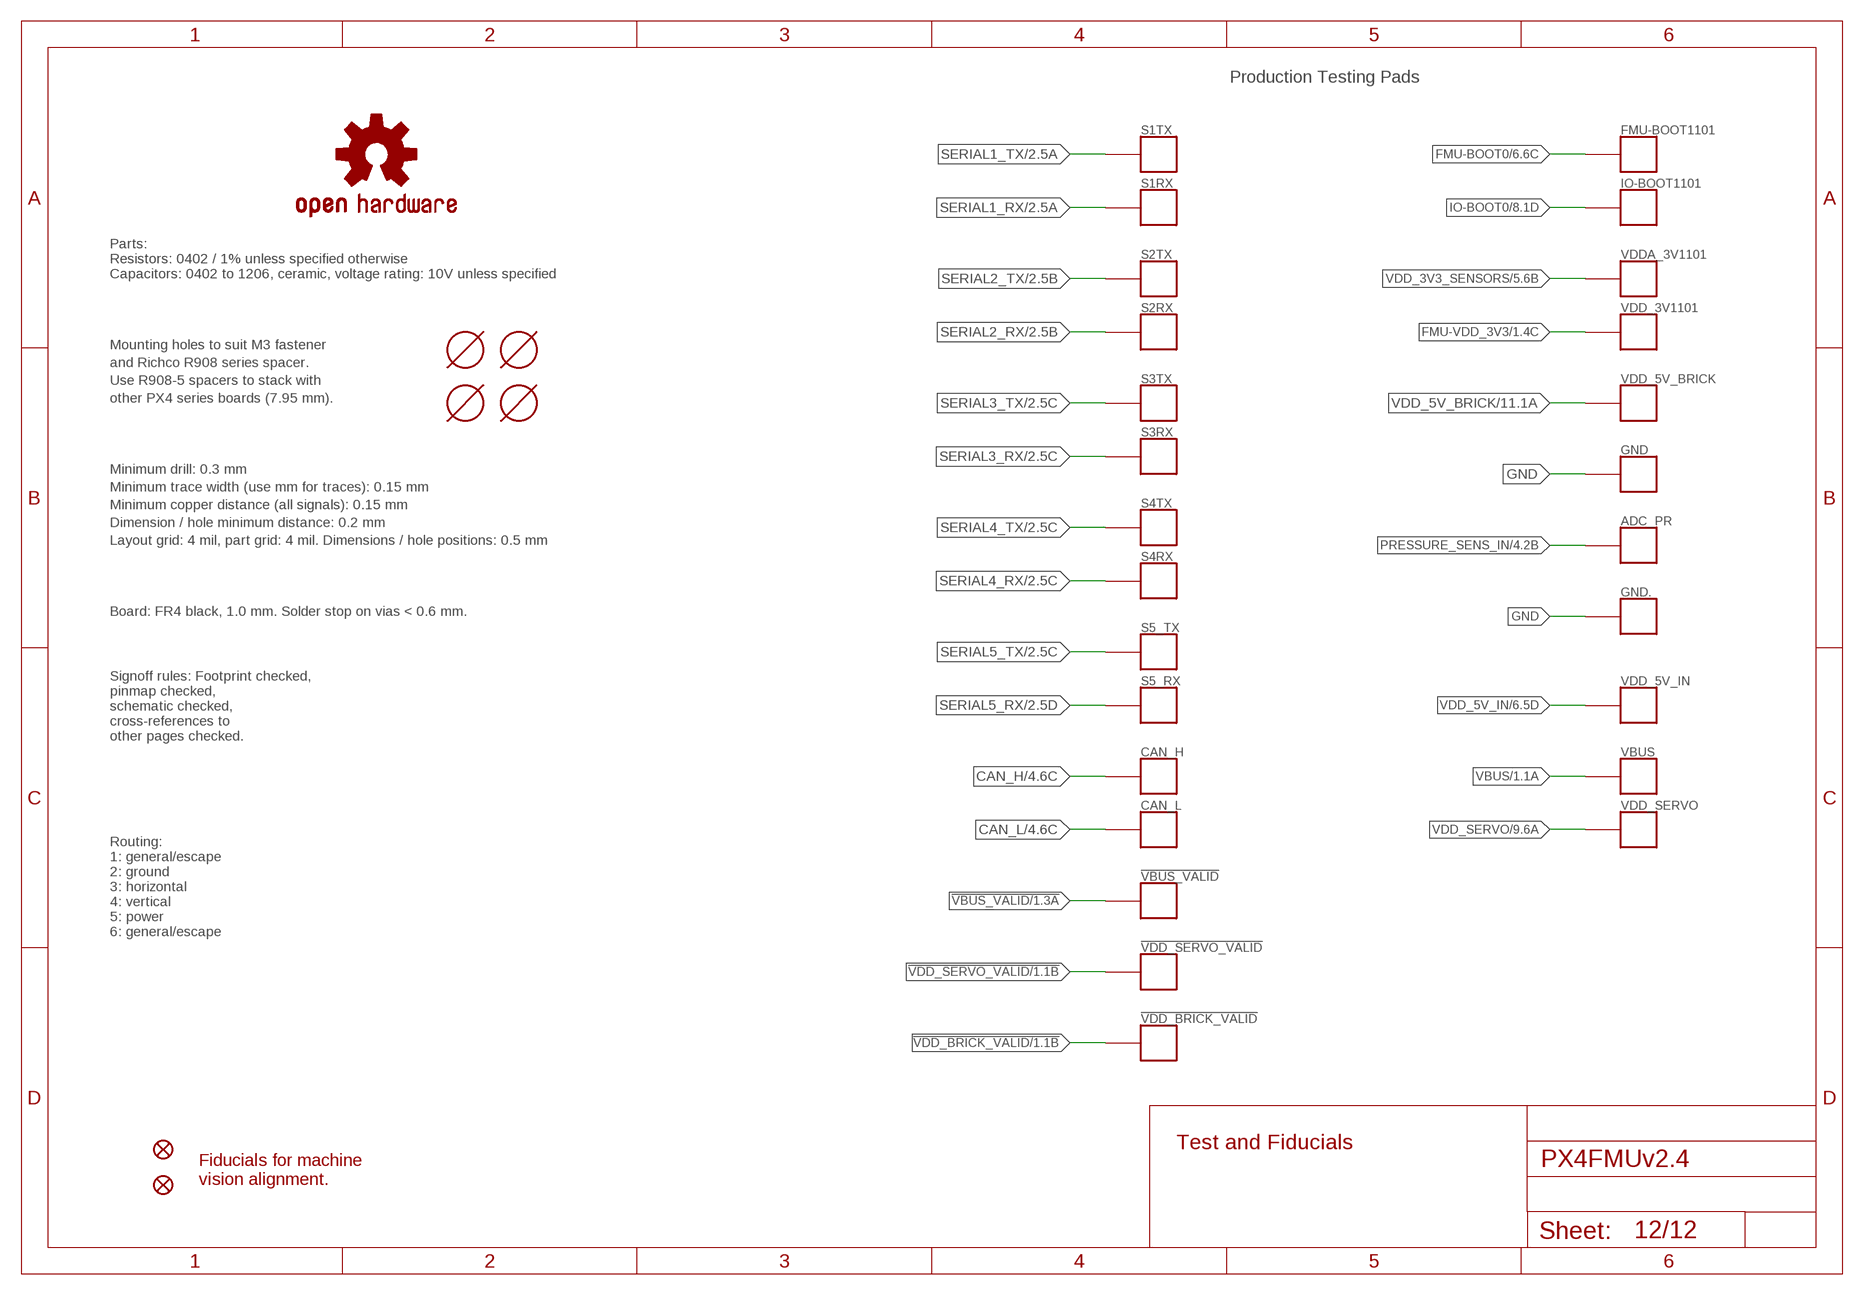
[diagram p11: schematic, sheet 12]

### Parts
!VBUS_VALID  PAD.04  [PAD.04X.04]
!VDD_BRICK_VALID  PAD.04  [PAD.04X.04]
!VDD_SERVO_VALID  PAD.04  [PAD.04X.04]
ADC_PR  PAD.04  [PAD.04X.04]
CAN_H  PAD.04  [PAD.04X.04]
CAN_L  PAD.04  [PAD.04X.04]
FMU-BOOT1101  PAD.04  [PAD.04X.04]
GND  PAD.04  [PAD.04X.04]
GND.  PAD.04  [PAD.04X.04]
IO-BOOT1101  PAD.04  [PAD.04X.04]
JP1  FIDUCIAL1.5X3  [FIDUCIAL-1.5X3]
JP2  FIDUCIAL1.5X3  [FIDUCIAL-1.5X3]
M3_MOUNT1101  MOUNT-HOLE3.1MM  [MOUNT-HOLE3.1]
M3_MOUNT1102  MOUNT-HOLE3.1MM  [MOUNT-HOLE3.1]
M3_MOUNT1103  MOUNT-HOLE3.1MM  [MOUNT-HOLE3.1]
M3_MOUNT1104  MOUNT-HOLE3.1MM  [MOUNT-HOLE3.1]
OSHW_LOGO  OSHW-LOGOS  [OSHW-LOGO-S]
S1RX  PAD.04  [PAD.04X.04]
S1TX  PAD.04  [PAD.04X.04]
S2RX  PAD.04  [PAD.04X.04]
S2TX  PAD.04  [PAD.04X.04]
S3RX  PAD.04  [PAD.04X.04]
S3TX  PAD.04  [PAD.04X.04]
S4RX  PAD.04  [PAD.04X.04]
S4TX  PAD.04  [PAD.04X.04]
S5_RX  PAD.04  [PAD.04X.04]
S5_TX  PAD.04  [PAD.04X.04]
VBUS  PAD.04  [PAD.04X.04]
VDD_3V1101  PAD.04  [PAD.04X.04]
VDD_5V_BRICK  PAD.04  [PAD.04X.04]
VDD_5V_IN  PAD.04  [PAD.04X.04]
VDD_SERVO  PAD.04  [PAD.04X.04]
VDDA_3V1101  PAD.04  [PAD.04X.04]

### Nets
!VBUS_VALID: !VBUS_VALID.P$1 ; also sheet 1,11
!VDD_BRICK_VALID: !VDD_BRICK_VALID.P$1 ; also sheet 1,11
!VDD_SERVO_VALID: !VDD_SERVO_VALID.P$1 ; also sheet 1,11
CAN_H: CAN_H.P$1 ; also sheet 4
CAN_L: CAN_L.P$1 ; also sheet 4
FMU-BOOT0: FMU-BOOT1101.P$1 ; also sheet 6
FMU-VDD_3V3 [power]: VDD_3V1101.P$1 ; also sheet 1,2,3,4,6,7,9
GND [power]: GND..P$1 GND.P$1 ; also sheet 1,2,3,4,5,6,7,8,9,10,11
IO-BOOT0: IO-BOOT1101.P$1 ; also sheet 8
PRESSURE_SENS_IN: ADC_PR.P$1 ; also sheet 4
SERIAL1_RX: S1RX.P$1 ; also sheet 2
SERIAL1_TX: S1TX.P$1 ; also sheet 2
SERIAL2_RX: S2RX.P$1 ; also sheet 2
SERIAL2_TX: S2TX.P$1 ; also sheet 2
SERIAL3_RX: S3RX.P$1 ; also sheet 2
SERIAL3_TX: S3TX.P$1 ; also sheet 2
SERIAL4_RX: S4RX.P$1 ; also sheet 2
SERIAL4_TX: S4TX.P$1 ; also sheet 2
SERIAL5_RX: S5_RX.P$1 ; also sheet 2
SERIAL5_TX: S5_TX.P$1 ; also sheet 2
VBUS [power]: VBUS.P$1 ; also sheet 1,3,11
VDD_3V3_SENSORS [power]: VDDA_3V1101.P$1 ; also sheet 5,6
VDD_5V_BRICK [power]: VDD_5V_BRICK.P$1 ; also sheet 11
VDD_5V_IN [power]: VDD_5V_IN.P$1 ; also sheet 6,7,10,11
VDD_SERVO [power]: VDD_SERVO.P$1 ; also sheet 9,11

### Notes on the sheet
- Production Testing Pads
- Parts:
  Resistors: 0402 / 1% unless specified otherwise
  Capacitors: 0402 to 1206, ceramic, voltage rating: 10V unless specified
- Mounting holes to suit M3 fastener
- and Richco R908 series spacer.
- Use R908-5 spacers to stack with
- other PX4 series boards (7.95 mm).
- Minimum drill: 0.3 mm
- Minimum trace width (use mm for traces): 0.15 mm
- Minimum copper distance (all signals): 0.15 mm
- Dimension / hole minimum distance: 0.2 mm
- Layout grid: 4 mil, part grid: 4 mil. Dimensions / hole positions: 0.5 mm
- Board: FR4 black, 1.0 mm. Solder stop on vias < 0.6 mm.
- Signoff rules: Footprint checked,
  pinmap checked,
  schematic checked, 
  cross-references to
  other pages checked.
- Routing:
  1: general/escape
  2: ground
  3: horizontal
  4: vertical
  5: power
  6: general/escape
- Test and Fiducials
- Fiducials for machine
  vision alignment.

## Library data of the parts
!VBUS_VALID !VDD_BRICK_VALID !VDD_SERVO_VALID ADC_PR CAN_H CAN_L FMU-BOOT1101 GND GND. IO-BOOT1101 S1RX S1TX S2RX S2TX S3RX S3TX S4RX S4TX S5_RX S5_TX VBUS VDD_3V1101 VDD_5V_BRICK VDD_5V_IN VDD_SERVO VDDA_3V1101 = pixhawk2:PAD: Test pad; BOM: EXCLUDE; PARTNO: *
B601 = pixhawk2:MS621FE: SEIKO 6.8mm Rechargeable 3V lithium battery; DATASHEET: http://speed.sii.co.jp/data/file_PRODUCT_MASTER_50112_TITLE_IMAGESP.pdf; LINK: http://search.digikey.com/us/en/products/MS621FE-FL11E/728-1057-ND/1889208; MFGPN: MS621FE; PARTNO: MS621FE-FL11E
C101 C201 C202 C401 C402 C502 C503 C507 C508 C512-C514 C606-C610 C612 C615-C617 C701 C801-C804 C901-C903 C1005 C1105-C1107 = pixhawk2:CAP: Capacitor; PARTNO: CC0402ZRY5V7BB104
C102 C103 C805 C806 = pixhawk2:CAP: Capacitor; PARTNO: C1005C0G1H080C
C501 C506 C509 C511 = pixhawk2:CAP: Capacitor; PARTNO: CC0805ZKY5V6BB106
C504 C505 C602 C1002 = pixhawk2:CAP: Capacitor; PARTNO: CC0402KRX7R7BB103
C510 C704 = pixhawk2:CAP: Capacitor; PARTNO: C1005X5R1C474K050BC
C515 = pixhawk2:CAP: Capacitor; PARTNO: GRM155R71E103JA01J
C601 C1001 = pixhawk2:CAP: Capacitor; PARTNO: CL21A106KAYNNNE
C603 C702 C1003 C1004 C1008 = pixhawk2:CAP: Capacitor; PARTNO: CC0603ZRY5V7BB105
C604 C605 C1101-C1103 = pixhawk2:CAP: Capacitor; PARTNO: CL21A226MAQNNNE
C611 C613 = pixhawk2:CAP: Capacitor; PARTNO: C1608Y5V1C225Z
C614 C618 C1104 = pixhawk2:CAP: Capacitor; PARTNO: C3216X5R1A107M160AC
C703 = pixhawk2:CAP: Capacitor; PARTNO: CC0402KRX7R7BB562
C1108-C1110 = pixhawk2:CAP: Capacitor; PARTNO: GRM1555C1E102JA01D
D1 = pixhawk2:DIODE-SCHOTTKY: Schottky barrier diode in DO214AC, e.g. Fairchild SS14.; PARTNO: MSS1P4-M3/89A
D2 = pixhawk2:DIODE-SCHOTTKY: Schottky barrier diode in DO214AC, e.g. Fairchild SS14.; PARTNO: RB751V40T1G
D201-D203 D401-D404 D701 D801 D901-D903 = pixhawk2:DIODE-TVS; PARTNO: PESD0402-140
D1001 = pixhawk2:PMEG2005CT: 500 mA low VF dual MEGA Schottky barrier rectifier http://www.nxp.com/documents/data_sheet/PMEG2005CT.pdf; PARTNO: PMEG2005CT
F1001 = pixhawk2:PTC: Resettable Fuse PTC; PARTNO: 0ZCA0035FF2G
J201-J204 J601 = con-hirose-df13:DF13-6P-1.25: DF13-6P 1.25mm Pitch Miniature Crimping Connector.; PARTNO: DF13C-6P-1.25V(20)
J301 = pixhawk2:MOLEX-47346-0001: MICRO USB B, BOTTOM MOUNT; PARTNO: 47346-0001
J302 J401 J405 = con-hirose-df13:DF13-4P-1.25: DF13-4P 1.25mm Pitch Miniature Crimping Connector.; PARTNO: DF13C-4P-1.25V(20)
J402 J702 = con-hirose-df13:DF13-3P-1.25: DF13-3P 1.25mm Pitch Miniature Crimping Connector.; PARTNO: DF13C-3P-1.25V(20)
J403 = con-hirose-df13:DF13-7P-1.25: DF13-7P 1.25mm Pitch Miniature Crimping Connector.; PARTNO: DF13C-7P-1.25V(20)
J404 = con-hirose-df13:DF13-5P-1.25: DF13-5P 1.25mm Pitch Miniature Crimping Connector.; PARTNO: DF13C-5P-1.25V(20)
J701 = con-hirose-df13:DF13-2P-1.25: DF13-2P; PARTNO: DF13C-2P-1.25V(20)
J801 = for-transfers:JST-ZH-3; PARTNO: B3B-ZR-SM4-TF (LF)(SN)(P)
J901 = pixhawk2:HEADER-3X16: 3x16 servo header; BOM: EXCLUDE
JP1 JP2 = pixhawk2:FIDUCIAL: Fiducial Alignment Points; BOM: EXCLUDE; PARTNO: *
JX301 JX802 = pixhawk2:ARM_MINI_JTAG: CONNECTOR wire to board 1.25 mm (.049 inch) pitch header; BOM: EXCLUDE; PARTNO: M50-3900542
JX801 = pixhawk2:HEADER-3X1: Single row 0.1" servo header; BOM: EXCLUDE
L201-L203 L401-L404 L603 L901 L1101 L1102 = pixhawk2:KNH16C104DA5TS: Kyocera KNH16C104DA5TS EMI filter; PARTNO: KNH16C104DA5TS
L701 = pixhawk2:INDUCTOR: Inductors; PARTNO: MLZ2012M470W
LED701 LED703 = pixhawk2:LED: LEDs; PARTNO: APTD1608SECK
LED702 LED704 = pixhawk2:LED: LEDs; PARTNO: APTD1608CGCK
LED705 = pixhawk2:LED: LEDs; PARTNO: APTD1608QBC/D
M3_MOUNT1101-M3_MOUNT1104 = pixhawk2:MOUNT-HOLE; BOM: EXCLUDE; PARTNO: *
OSHW_LOGO = pixhawk2:OSHW-LOGO: Open Source Hardware Logo This logo indicates the piece of hardware it is found on incorporates a OSHW license and/or adheres to the definition of open source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; BOM: EXCLUDE; PARTNO: *
Q601 = transistor-pnp:MMBT3906*: PNP Transistror; PARTNO: MMBT 3906 LT1
R3 R4 R707-R709 R711 R712 R803 R804 R902-R917 = pixhawk2:RESISTOR: Resistor; PARTNO: RC0402FR-07220RL
R101 = pixhawk2:RESISTOR: Resistor; PARTNO: RC0402FR-07470RL
R102 R611 R615 R635 R702 R704 R801 R802 R901 R1002 = pixhawk2:RESISTOR: Resistor; PARTNO: RC0402FR-0710KL
R201-R216 R404 R405 R409 = pixhawk2:RESISTOR: Resistor; PARTNO: RC0402FR-07120RL
R301-R305 R703 R1001 = pixhawk2:RESISTOR: Resistor; PARTNO: RC0402FR-07100KL
R306 R307 R401 R402 R713 = pixhawk2:RESISTOR: Resistor; PARTNO: RC0402FR-071K5L
R403 R406-R408 R609 R610 R918 R919 R922 R1101 R1102 = pixhawk2:RESISTOR: Resistor; PARTNO: ERA-2AEB103X
R602 R604 R1103 R1104 = pixhawk2:RESISTOR: Resistor; PARTNO: RC0402FR-071ML
R603 = pixhawk2:RESISTOR: Resistor; BOM: EXCLUDE; PARTNO: RC0402FR-0710KL
R608 = pixhawk2:RESISTOR: Resistor; PARTNO: RC0402FR-071KL
R616 = pixhawk2:RESISTOR: Resistor; PARTNO: RMCF0402FT25K5
R617 R706 = pixhawk2:RESISTOR: Resistor; PARTNO: RMCF0402FT16K5
R620 = pixhawk2:RESISTOR: Resistor; PARTNO: RC1005F182CS
R621 = pixhawk2:RESISTOR: Resistor; PARTNO: RC1608J100CS
R701 = pixhawk2:RESISTOR: Resistor; PARTNO: RMCF0402FT9K09
R705 R1105 R1109 R1112 = pixhawk2:RESISTOR: Resistor; PARTNO: RMCF0402FT453K
R710 = pixhawk2:RESISTOR: Resistor; PARTNO: ERJ-2GEJ680X
R1106 R1110 R1113 = pixhawk2:RESISTOR: Resistor; PARTNO: ERA-2AEB563X
R1107 R1111 R1114 = pixhawk2:RESISTOR: Resistor; PARTNO: ERJ-2RKF1053X
R1115 = pixhawk2:RESISTOR: Resistor; PARTNO: ERJ-2GE0R00X
RN1101 = resistor-dil:4R-N: Array Chip Resistor Source: RS Component / Phycomp; OC_FARNELL: unknown; OC_NEWARK: unknown; PARTNO: EXB-28V105JX
S601 S801 = pixhawk2:SWITCH-MOMENTARY-2; PARTNO: EVQP7J01K
U101 = pixhawk2:STM32F4X7VX: STM32F4X7VX 100 pin LQFP STM32F407VE - 512 KB flash, no crypto STM32F407VG - 1 MB flash, no crypto STM32F417VE - 512 KB flash, with crypto STM32F417VG - 1 MB flash, with crypto; PARTNO: STM32F427VI
U102 = pixhawk2:FM25V01: FM25V01 128Kb Serial 3V F-RAM Memory; DATASHEET: http://www.ramtron.com/files/datasheets/FM25V01_ds.pdf; LINK: http://www.digikey.com/product-detail/en/FM25V01-GTR/1140-1026-1-ND/2809832; MFGPN: FM25V01; PARTNO: FM25V01-G
U201 U202 U901 U902 = pixhawk2:TXS0108; PARTNO: TXS0108ERGYR
U301 = baseboard:MICROSDSDI; PARTNO: 2908-05WB-MG
U302 = pixhawk2:NUF2042XV6; PARTNO: NUF2042XV6T1G
U401 = pixhawk2:MAX3051: 3.3-V CAN TRANSCEIVER; PARTNO: MAX3051EKA
U501 = pixhawk2:L3G4200DH: L3G4200DH - Digital 3-axis Gyroscope The L3G4200DH is a low-power three-axis angular rate sensor. The L3G4200DH has a full scale of ±250/±500/ ±2000 dps and is capable of measuring rates with a user-selectable bandwidth. It can operate within a temperature range from -40 °C to +85 °C. Supply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; PARTNO: L3GD20
U502 = pixhawk2:L3GD20H: L3GD20H MEMS motion sensor: 3-axis digital output gyroscope; BOM: EXCLUDE; DATASHEET: http://www.st.com/internet/com/TECHNICAL_RESOURCES/TECHNICAL_LITERATURE/DATASHEET/DM00060659.pdf; LINK: http://www.st.com/internet/analog/product/254039.jsp; MFGPN: L3GD20H; PARTNO: L3GD20H
U504 = pixhawk2:LSM303D: LSM303D Ultra compact high performance e-compass: 3D accelerometer and 3D magnetometer module; DATASHEET: http://www.st.com/internet/com/TECHNICAL_RESOURCES/TECHNICAL_LITERATURE/DATASHEET/DM00057547.pdf; LINK: http://www.st.com/internet/analog/product/253884.jsp; MFGPN: LSM303D; PARTNO: LSM303D
U505 = pixhawk2:MPU-6000: Invensense MPU-6000: 3-axis gyro, 3-axis accel & 9-axis MotionFusion The MPU-60X0 Motion Processing Unit (MPU?) is the world?s first motion processing solution with integrated 9-axis sensor fusion for handset and tablet applications, game controllers, motion pointer remote controls, and other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; DATASHEET: http://invensense.com/mems/gyro/documents/PS-MPU-6000A-00_v1.0.pdf; LINK: http://invensense.com/mems/gyro/mpu6000.html; MFGPN: MPU-6000; PARTNO: MPU-6000
U506 = pixhawk2:MS5611-01BA: MS5611-01BA The MS5611-01BA is a new generation of high resolution altimeter sensors from MEAS Switzerland with SPI and I 2 C bus interface. It is optimized for altimeters and variometers with an altitude resolution of 10 cm. The sensor module includes a high linearity pressure sensor and an ultra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; DATASHEET: http://www.meas-spec.com/downloads/MS5611-01BA01.pdf; LINK: http://www.meas-spec.com/product/t_product.aspx?id=8503#; MFGPN: MS5611-01BA; PARTNO: MS5611-01BA
U601 U602 = pixhawk2:BQ24315; PARTNO: BQ24315DSGR
U603 U1002 = pixhawk2:MIC5332; PARTNO: MIC5332-SSYMT
U701 = pixhawk2:TCA62724FMG: Toshiba TCA62724FMG I2C RGB LED driver; PARTNO: TCA62724FMG
U702 = pixhawk2:LT3469: LT3469 Piezo microactuator driver with boost regulator; PARTNO: LT3469ETS8
U703 = pixhawk2:RGB-LED: RGB LED with separate anode/cathode terminals; PARTNO: LRTB GFTG-T7AW-1+V7A7-29+R5T9-49-L
U801 = pixhawk2:STM32F10XCXT6: ST STM32F101/103 48pin LQFP; PARTNO: STM32F100C8T6B
U903 = pixhawk2:74LVC2G240: Dual inverter tri-state, 3.3V/5V compatible http://www.nxp.com/documents/data_sheet/74LVC2G240.pdf http://focus.ti.com/lit/ds/symlink/sn74lvc2g240.pdf; PARTNO: 74LVC2G240DP,125
U1001 = pixhawk2:BQ24313; PARTNO: BQ24313DSGT
U1101 = pixhawk2:LTC4117; PARTNO: LTC4417IUF#PBF
U1102-U1104 = pixhawk2:MOSFET-DUAL-PCHANNEL; PARTNO: NTHD4102PT1G
X101 X801 = pixhawk2:OSCILLATOR: Crystal Oscillator in 3.2x2.5 SMD; PARTNO: NX3225SA-24.000000MHZ
X503 = pixhawk2:CONN_FPC_10: 10-pin FPC connector for PX4 sensor board; PARTNO: 0781191109

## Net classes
0 signal: width 0.15 mm, drill 0.15 mm, clearance 0.152 mm
1 power: width 0.15 mm, drill 0.2 mm, clearance 0.152 mm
